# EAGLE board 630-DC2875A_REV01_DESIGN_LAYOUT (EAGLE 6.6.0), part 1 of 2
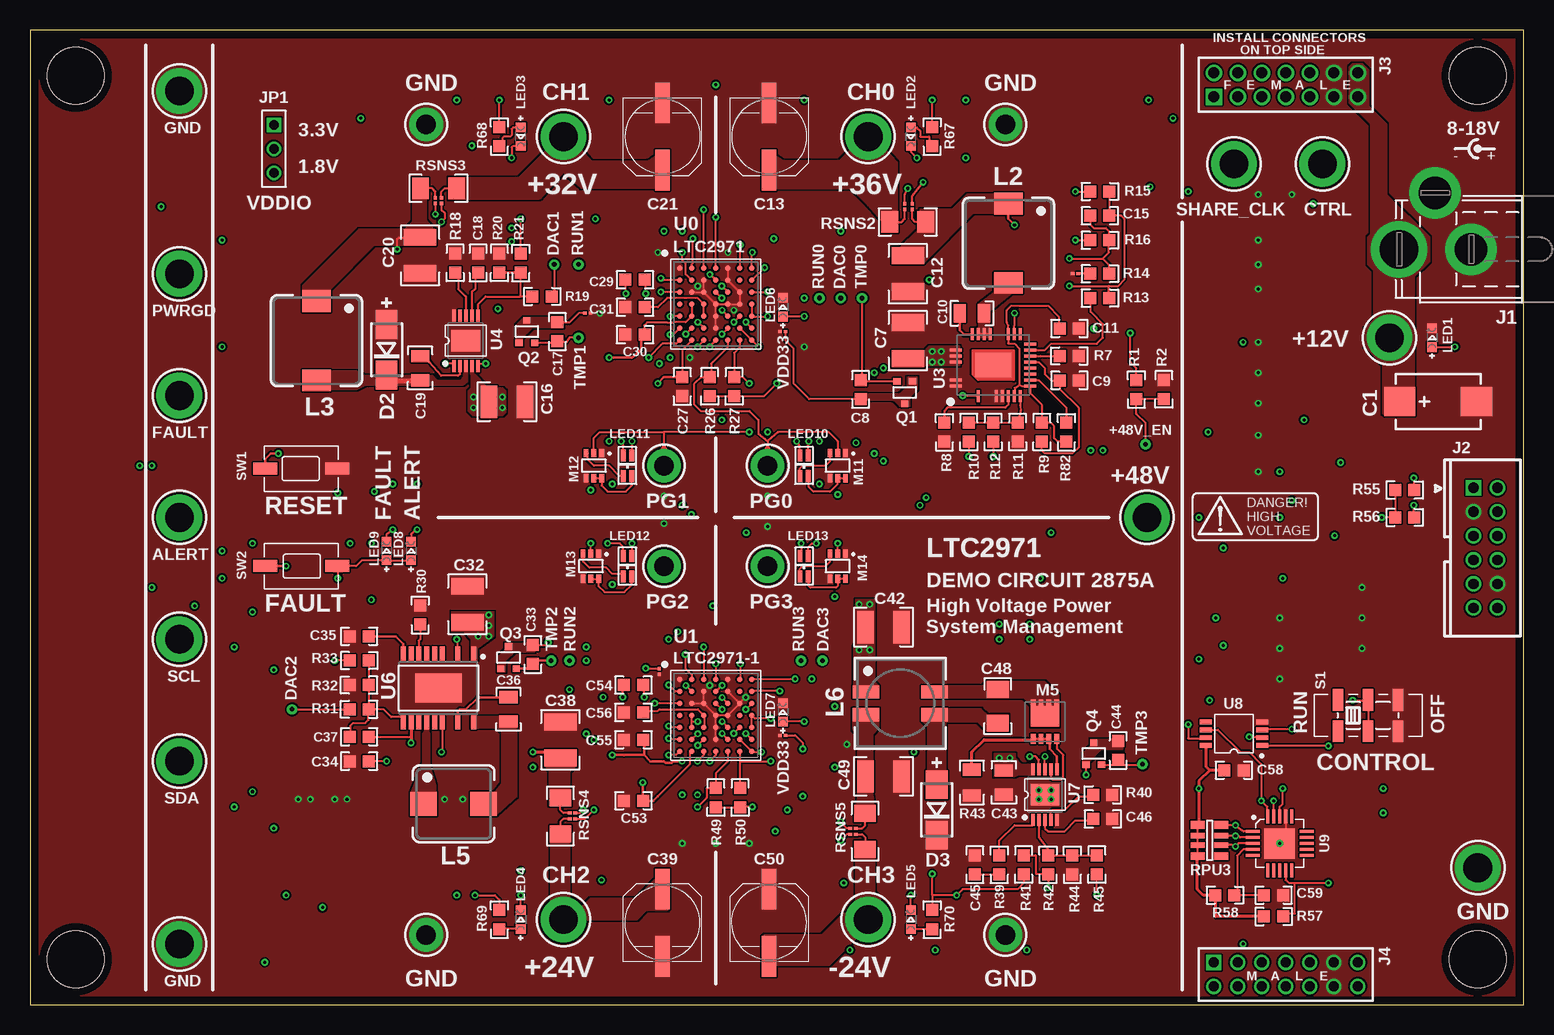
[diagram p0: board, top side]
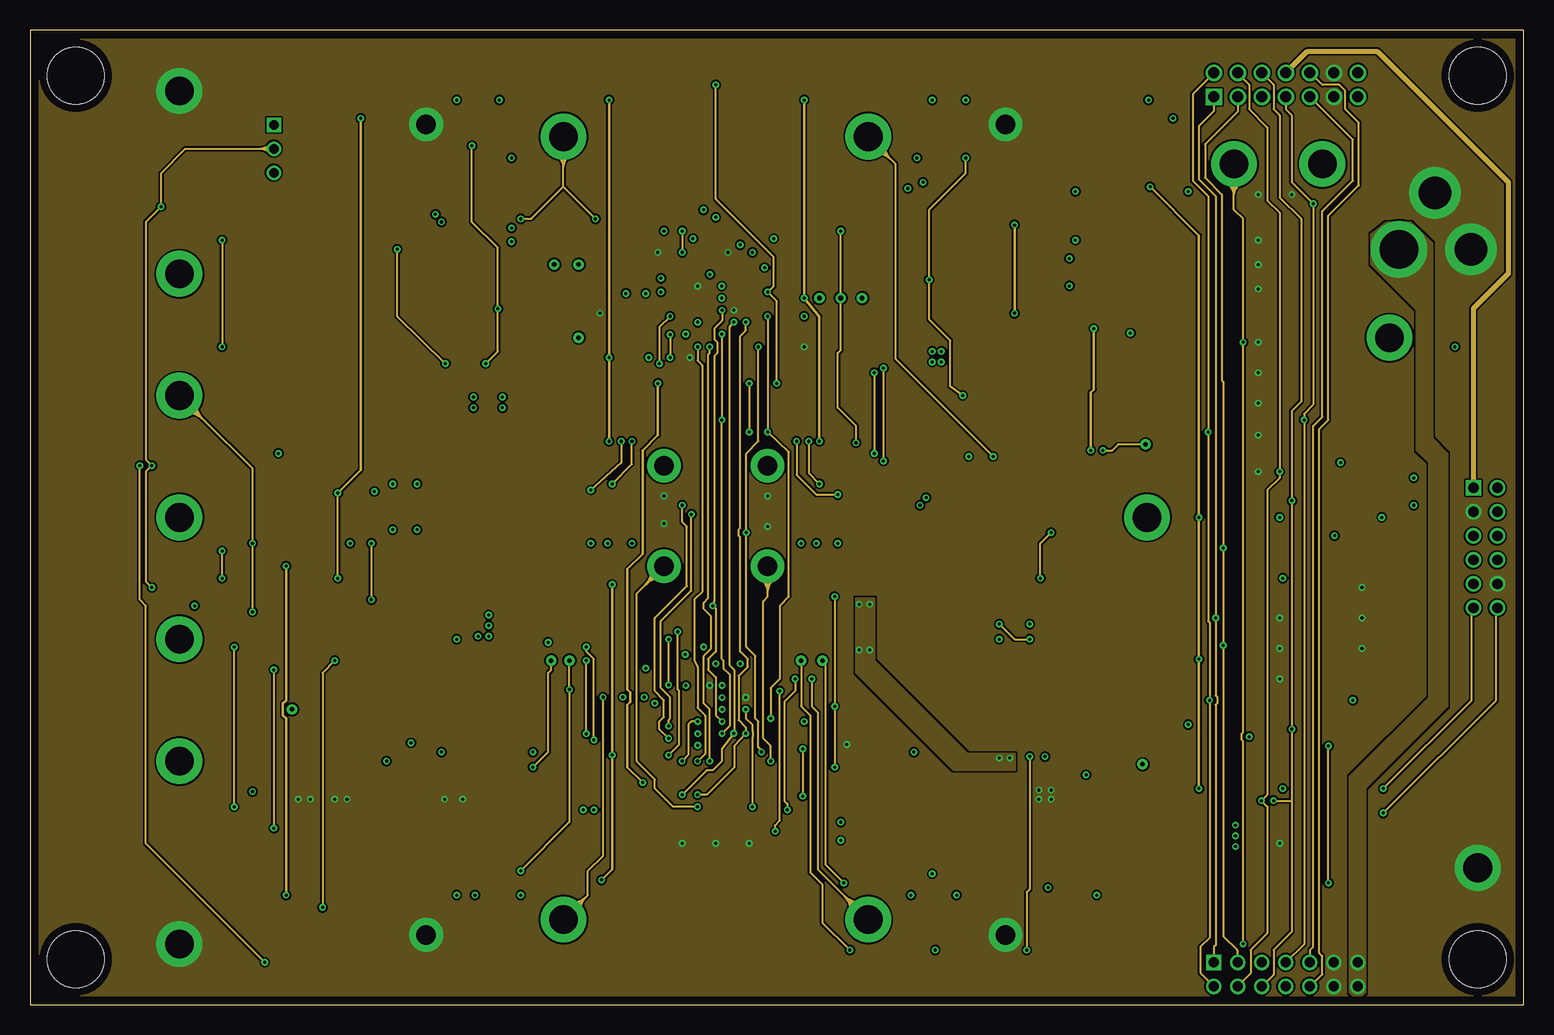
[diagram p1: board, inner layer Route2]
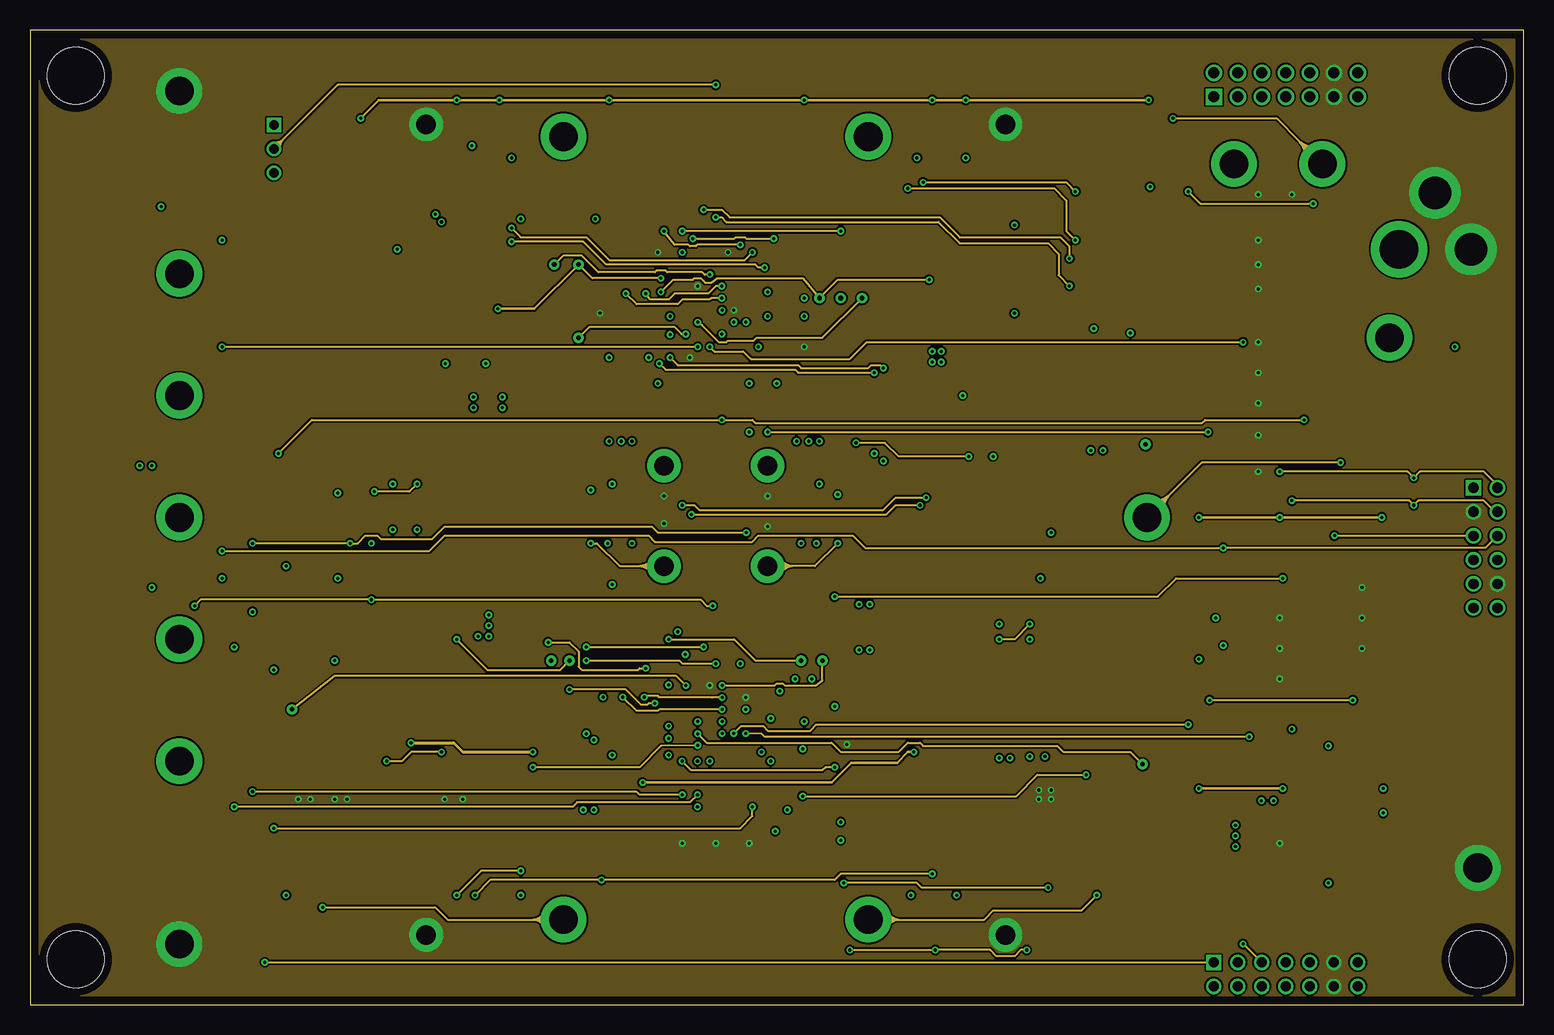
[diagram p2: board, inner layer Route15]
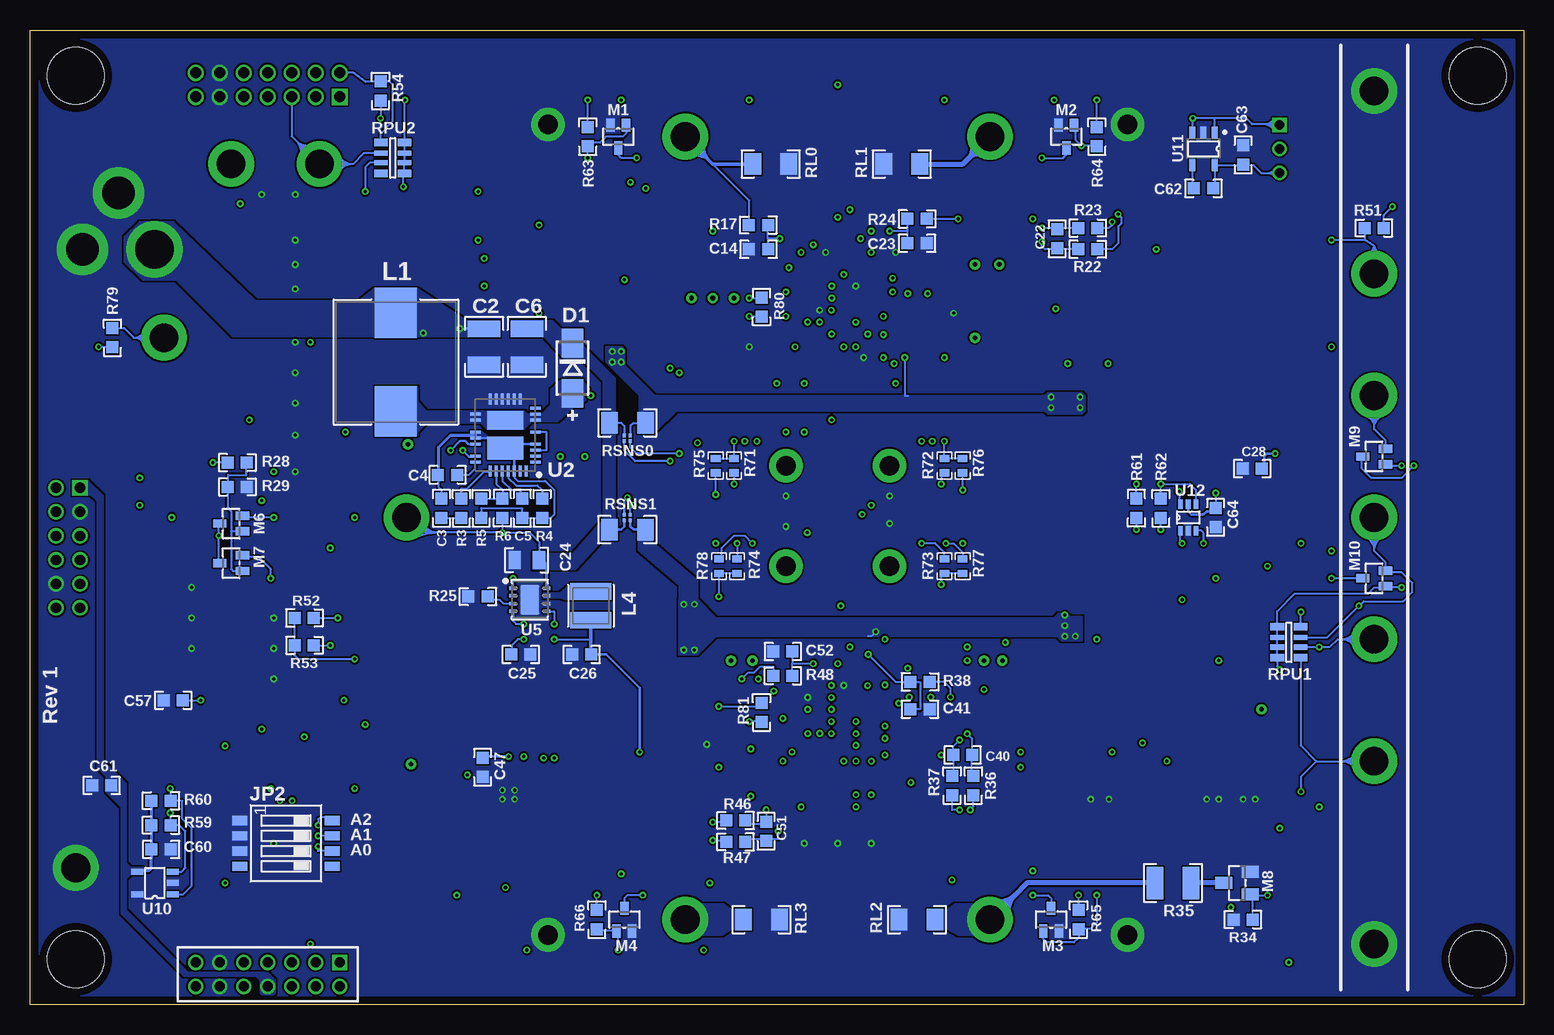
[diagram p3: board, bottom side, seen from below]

Size 124.46 x 81.28 mm. Coordinates in mm from the lower left corner, seen from the top.
Outline: 0,0 124.46,0 124.46,81.28 0,81.28 0,0
Copper layers (1*2+15*16): Top 0.035mm / dielectric 0.11mm / Route2 0.035mm / dielectric 1.13mm / Route15 0.035mm / dielectric 0.11mm / Bottom 0.035mm
Design rules "default *": minimum track width 6mil, minimum drill 10mil, track to track 6mil, track to pad 6mil, pad to pad 6mil, via to via 6mil, smd to smd 4mil, copper to edge 25mil, drill to drill 20mil, minimum pad ring 6mil, minimum via ring 6mil, stop-mask expansion 4mil, vias tented up to drill 15mil, thermal gap 10mil
Net classes: 1 HV: clearance 0.178 mm
Holes 4.75 mm at 3.81,3.81 3.81,77.47 120.65,77.47 120.65,3.81

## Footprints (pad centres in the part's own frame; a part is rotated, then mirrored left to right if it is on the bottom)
C7343 = smd 2.6 x 2.4: + -3.2,0; - 3.2,0
C1210_BOX = smd 1.4 x 2.7: 1 -1.5,0; 2 1.5,0
C0603_BOX = smd 1 x 1: 1 -0.8,0; 2 0.8,0
C0805_BOX = smd 1.016 x 1.524: 1 -1.016,0; 2 1.016,0
UD-6,3X5,8_NICHICON = smd 3.4 x 1.2: + 2.8,0; - -2.8,0
C1206_BOX = smd 1.4 x 1.8: 1 -1.4,0; 2 1.4,0
SMA = smd 2.4 x 1.8: A 2.1,0; C -2.1,0
PJ-002A/B = drill 3.2 pad 4.7: 1 3,0 | drill 2.7 pad 4.3: 2 -3,0; 3 0,-4.7
CONN_DC1613 = drill 0.86 square: 1 -5,-1 | drill 0.86: 2 -5,1; 3 -3,-1; 4 -3,1; 5 -1,-1; 6 -1,1; 7 1,-1; 8 1,1; 9 3,-1; 10 3,1; 11 5,-1; 12 5,1
2X07M = drill 0.914 square: 1 -6,-1 | drill 0.914: 2 -6,1; 3 -4,-1; 4 -4,1; 5 -2,-1; 6 -2,1; 7 0,-1; 8 0,1; 9 2,-1; 10 2,1; 11 4,-1; 12 4,1; 13 6,-1; 14 6,1
2X07M' = drill 0.85 square: 1 -6,-1 | drill 0.85: 2 -6,1; 3 -4,-1; 4 -4,1; 5 -2,-1; 6 -2,1; 7 0,-1; 8 0,1; 9 2,-1; 10 2,1; 11 4,-1; 12 4,1; 13 6,-1; 14 6,1
1X03-2MM = drill 0.8 square: 1 -2,0 | drill 0.8: 2 0,0; 3 2,0
SMT_DIP_4 = smd 1.27 x 0.762: 1 -3.861,1.905; 2 -3.861,0.635; 3 -3.861,-0.635; 4 -3.861,-1.905; 5 3.861,-1.905; 6 3.861,-0.635; 7 3.861,0.635; 8 3.861,1.905
WE-LHMI-10 = smd 4.2 x 3.5: 1 -4.1,0; 2 4.1,0
WE-PD-7.3 = smd 1.8 x 2.4: 1 3.3,0; 2 -3.3,0
WE-MAPI-3015 = smd 1.4 x 3.4: 1 -1.2,0; 2 1.2,0
WE-PD-6.0 = smd 2.2 x 2: 1 2.5,0; 2 -2.5,0
WE-DD-7.3 = smd 2.2 x 1.1: 1 -2.85,0.95; 2 -2.85,-0.95; 3 2.85,-0.95; 4 2.85,0.95
CHIPLED_0603 = smd 0.8 x 0.8: A -0.78,0; C 0.78,0
LED-DUAL_1.6X0.8MM = smd 1 x 0.4: 1 0.85,-0.35; 2 -0.85,-0.35; 3 0.85,0.35; 4 -0.85,0.35
SOT323 = smd 0.7 x 1.1: 1 -0.65,-0.95; 2 0.65,-0.95; 3 0,0.95
MLP-8 = smd 0.8 x 0.4: 1 -1.45,0.975; 2 -1.45,0.325; 3 -1.45,-0.325; 4 -1.45,-0.975 | smd 0.9 x 0.4: 5 1.4,-0.975; 6 1.4,-0.325; 7 1.4,0.325; 8 1.4,0.975 | smd 1.7 x 2.35: PAD 0.45,0
SOT23 = smd 1 x 1.4: 1 -0.95,-1.1; 2 0.95,-1.1; 3 0,1.1
SOT-363 = smd 0.7 x 0.4: 1 -1.05,0.65; 2 -1.05,0; 3 -1.05,-0.65; 4 1.05,-0.65; 5 1.05,0; 6 1.05,0.65
NODE_BREAKER = smd 0.305 x 0.254: 1 -0.229,0; 2 0.229,0
NODE_BREAKER_BOT = smd 0.305 x 0.254: 1 -0.229,0; 2 0.229,0
SC70 = smd 0.6 x 0.55: 1 -0.65,-0.925; 2 0.65,-0.925; 3 0,0.925
R0603_BOX = smd 1 x 1: 1 -0.8,0; 2 0.8,0
R1210_BOX = smd 1.4 x 2.7: 1 -1.5,0; 2 1.5,0
R0805_BOX = smd 1.016 x 1.524: 1 -1.077,0; 2 1.077,0
R0402_BOX = smd 0.6 x 0.8: 1 -0.6,0; 2 0.6,0
R1206_BOX = smd 1.4 x 1.8: 1 -1.5,0; 2 1.5,0
R_VISHAY_CRA06S = smd 1.15 x 0.63: R1_1 -0.975,1.295; R1_2 0.975,1.295; R4_1 -0.975,-1.295; R4_2 0.975,-1.295 | smd 1.15 x 0.44: R2_1 -0.975,0.4; R2_2 0.975,0.4; R3_1 -0.975,-0.4; R3_2 0.975,-0.4
JCQN = smd 0.9 x 1.8: 1 -2.5,1.3; 2 0,1.3; 3 2.5,1.3; 4 -2.5,-1.3; 5 0,-1.3; 6 2.5,-1.3
SWITCH_PTS635 = smd 2 x 1: SW1 -3,0; SW2 3,0
TURRET_LARGE_2501 = drill 2.388 pad 3.81: TP 0,0
TURRET_SMALL_2308 = drill 1.626 pad 2.794: TP1 0,0
VIA = drill 0.381 pad 0.864: 1 0,0
BGA49 = smd 0.47 x 0.47: A1 -3,3; A2 -2,3; A3 -1,3; A4 0,3; A5 1,3; A6 2,3; A7 3,3; B1 -3,2; B2 -2,2; B3 -1,2; B4 0,2; B5 1,2; B6 2,2; B7 3,2; C1 -3,1; C2 -2,1; C3 -1,1; C4 0,1; C5 1,1; C6 2,1; C7 3,1; D1 -3,0; D2 -2,0; D3 -1,0; D4 0,0; D5 1,0; D6 2,0; D7 3,0; E1 -3,-1; E2 -2,-1; E3 -1,-1; E4 0,-1; E5 1,-1; E6 2,-1; E7 3,-1; F1 -3,-2; F2 -2,-2; F3 -1,-2; F4 0,-2; F5 1,-2; F6 2,-2; F7 3,-2; G1 -3,-3; G2 -2,-3; G3 -1,-3; G4 0,-3; G5 1,-3; G6 2,-3; G7 3,-3
QFN36-5X6 = smd 0.25 x 0.9: 1 -2.25,-2.5; 2 -1.75,-2.5; 3 -1.25,-2.5; 4 -0.75,-2.5; 6 0.25,-2.5; 8 1.25,-2.5; 9 1.75,-2.5; 10 2.25,-2.5; 20 1.75,2.5; 21 1.25,2.5; 23 0.25,2.5; 24 -0.25,2.5; 25 -0.75,2.5; 27 -1.75,2.5; 28 -2.25,2.5 | smd 0.9 x 0.25: 12 3,-1.25; 13 3,-0.75; 14 3,-0.25; 15 3,0.25; 16 3,0.75; 17 3,1.25; 30 -3,1.25; 31 -3,0.75; 32 -3,0.25; 33 -3,-0.25; 34 -3,-0.75; 35 -3,-1.25; 36 -3,-1.75 | smd 1.88 x 3: 37 -1.07,0 | smd 1.53 x 3: 38 1.24,0
QFN36-5X6-UHE = smd 0.25 x 1: 3 -1.25,-2.6; 6 0.25,-2.6; 7 0.75,-2.6; 8 1.25,-2.6; 9 1.75,-2.6; 10 2.25,-2.6; 19 2.25,2.6; 20 1.75,2.6; 21 1.25,2.6; 24 -0.25,2.6; 25 -0.75,2.6; 26 -1.25,2.6; 27 -1.75,2.6 | smd 1 x 0.25: 11 3.1,-1.75; 12 3.1,-1.25; 13 3.1,-0.75; 14 3.1,-0.25; 15 3.1,0.25; 16 3.1,0.75; 17 3.1,1.25; 18 3.1,1.75; 30 -3.1,1.25; 31 -3.1,0.75; 32 -3.1,0.25; 35 -3.1,-1.25; 36 -3.1,-1.75 | smd 3 x 2: 37 0,0
MSOP10_EXP = smd 0.3 x 1: 1 -1,-2.1; 2 -0.5,-2.1; 3 0,-2.1; 4 0.5,-2.1; 5 1,-2.1; 6 1,2.1; 7 0.5,2.1; 8 0,2.1; 9 -0.5,2.1; 10 -1,2.1 | smd 2.4 x 1.8: PAD 0,0
LFCSP8 = smd 0.3 x 0.7: 1 -0.975,-1.4; 2 -0.325,-1.4; 3 0.325,-1.4; 4 0.975,-1.4; 5 0.975,1.4; 6 0.325,1.4; 7 -0.325,1.4; 8 -0.975,1.4 | smd 2.42 x 1.56: EXP 0,0
TSSOP20EXP_HV = smd 1.2 x 0.42: 1 -2.85,2.925; 3 -2.85,1.625; 5 -2.85,0.325; 6 -2.85,-0.325; 7 -2.85,-0.975; 8 -2.85,-1.625; 9 -2.85,-2.275; 10 -2.85,-2.925; 11 2.85,-2.925; 12 2.85,-2.275; 13 2.85,-1.625; 14 2.85,-0.975; 15 2.85,-0.325; 16 2.85,0.325; 18 2.85,1.625; 20 2.85,2.925 | smd 2.4 x 3.86: EXP 0,0
MSOP-8 = smd 0.406 x 1.016: 1 -0.975,-2.35; 2 -0.325,-2.35; 3 0.325,-2.35; 4 0.975,-2.35; 5 0.975,2.35; 6 0.325,2.35; 7 -0.325,2.35; 8 -0.975,2.35
QFN20 = smd 1.143 x 0.254: 1 -2.25,1; 2 -2.25,0.5; 3 -2.25,0; 4 -2.25,-0.5; 5 -2.25,-1; 11 2.25,-1; 12 2.25,-0.5; 13 2.25,0; 14 2.25,0.5; 15 2.25,1 | smd 0.254 x 1.143: 6 -1,-2.25; 7 -0.5,-2.25; 8 0,-2.25; 9 0.5,-2.25; 10 1,-2.25; 16 1,2.25; 17 0.5,2.25; 18 0,2.25; 19 -0.5,2.25; 20 -1,2.25 | smd 2.54 x 2.54: PAD 0,0
SOT-23-5 = smd 1 x 0.5: 1 -1.491,0.95; 2 -1.491,0; 3 -1.491,-0.95; 4 1.491,-0.95; 5 1.491,0.95
SOT-23-5' = smd 1 x 0.5: 1 -1.35,0.95; 2 -1.35,0; 3 -1.35,-0.95; 4 1.35,-0.95; 5 1.35,0.95
SC70-6 = smd 0.4 x 0.8: 1 -0.65,-1.102; 2 0,-1.102; 3 0.65,-1.102; 4 0.65,1.102; 5 0,1.098; 6 -0.65,1.102

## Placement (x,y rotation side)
C1  22uF/25V  [C7343]  117.35,50.29 0 top
C2  10uF/25V  [C1210_BOX]  86.61,54.86 270 bottom
C3  4.7nF  [C0603_BOX]  90.17,41.4 90 bottom
C4  4.7uF  [C0603_BOX]  89.66,44.2 180 bottom
C5  47nF  [C0603_BOX]  83.44,41.4 270 bottom
C6  4.7uF/63V  [C1210_BOX]  83.06,54.86 270 bottom
C7  4.7uF/63V  [C1210_BOX]  73.15,55.37 90 top
C8  0.1uF  [C0603_BOX]  69.22,51.31 270 top
C9  47nF  [C0603_BOX]  86.61,52.07 0 top
C10  0.1uF/63V  [C0805_BOX]  78.49,57.66 0 top
C11  1uF  [C0603_BOX]  86.61,56.39 0 top
C12  10uF/50V  [C1210_BOX]  73.15,60.96 270 top
C13  10uF/50V  [UD-6,3X5,8_NICHICON]  61.59,72.39 270 top
C14  47nF/50V  [C0603_BOX]  63.75,62.99 180 bottom
C15  0.1uF  [C0603_BOX]  89.15,65.79 180 top
C16  4.7uF/63V  [C1210_BOX]  39.75,50.29 0 top
C17  0.1uF  [C0603_BOX]  43.94,56.13 90 top
C18  47nF  [C0603_BOX]  37.34,61.85 90 top
C19  0.22uF/63V  [C0805_BOX]  32.51,53.09 270 top
C20  10uF/50V  [C1210_BOX]  32.51,62.48 270 top
C21  10uF/50V  [UD-6,3X5,8_NICHICON]  52.7,72.39 270 top
C22  0.1uF  [C0603_BOX]  38.86,63.88 90 bottom
C23  47nF/50V  [C0603_BOX]  50.55,63.5 0 bottom
C24  1uF/63V  [C0805_BOX]  83.06,37.08 180 bottom
C25  2.2nF  [C0603_BOX]  83.57,29.21 0 bottom
C26  4.7uF/10V  [C0603_BOX]  78.49,29.21 180 bottom
C27  0.1uF  [C0603_BOX]  54.36,51.56 90 top
C28  10nF  [C0603_BOX]  22.61,44.7 0 bottom
C29  0.1uF  [C0603_BOX]  50.42,60.45 180 top
C30  0.1uF  [C0603_BOX]  50.42,55.88 180 top
C31  0.1uF  [C0603_BOX]  50.42,58.17 0 top
C32  4.7uF/63V  [C1210_BOX]  36.45,33.4 90 top
C33  0.1uF  [C0603_BOX]  41.91,29.21 90 top
C34  4.7uF/10V  [C0603_BOX]  27.43,20.32 180 top
C35  47nF  [C0603_BOX]  27.43,30.73 180 top
C36  0.1uF/63V  [C0805_BOX]  39.88,24.64 270 top
C37  22pF  [C0603_BOX]  27.43,22.35 180 top
C38  10uF/35V  [C1210_BOX]  44.2,22.1 90 top
C39  10uF/35V  [UD-6,3X5,8_NICHICON]  52.7,6.86 90 top
C40  0.1uF  [C0603_BOX]  46.74,20.83 180 bottom
C41  47nF/50V  [C0603_BOX]  50.29,24.64 0 bottom
C42  4.7uF/63V  [C1210_BOX]  71.12,31.5 0 top
C43  0.1uF/63V  [C0805_BOX]  81.15,18.54 270 top
C44  0.1uF  [C0603_BOX]  90.68,21.21 90 top
C45  4.7nF  [C0603_BOX]  78.74,11.68 90 top
C46  220nF  [C0603_BOX]  89.41,15.49 0 top
C47  4.7uF/10V  [C0603_BOX]  86.74,19.81 270 bottom
C48  2.2uF/100V  [C1206_BOX]  80.64,24.89 270 top
C49  10uF/35V  [C1210_BOX]  71.12,19.05 0 top
C50  10uF/35V  [UD-6,3X5,8_NICHICON]  61.59,6.86 90 top
C51  0.1uF  [C0603_BOX]  63.12,14.48 270 bottom
C52  47nF/50V  [C0603_BOX]  61.72,29.46 180 bottom
C53  0.1uF  [C0603_BOX]  50.29,17.02 180 top
C54  0.1uF  [C0603_BOX]  50.29,26.67 180 top
C55  0.1uF  [C0603_BOX]  50.29,22.1 180 top
C56  0.1uF  [C0603_BOX]  50.29,24.38 180 top
C57  1uF  [C0603_BOX]  112.52,25.4 180 bottom
C58  0.1uF  [C0603_BOX]  100.33,19.56 0 top
C59  1uF  [C0603_BOX]  103.63,9.14 0 top
C60  0.1uF  [C0603_BOX]  113.54,12.95 0 bottom
C61  1uF/10V  [C0603_BOX]  118.49,18.29 180 bottom
C62  10nF  [C0603_BOX]  26.67,68.07 180 bottom
C63  4.7uF/10V  [C0603_BOX]  23.37,70.87 90 bottom
C64  0.1uF  [C0603_BOX]  25.65,40.64 270 bottom
D1  B160-13-F  [SMA]  79.25,53.09 270 bottom
D2  B160-13-F  [SMA]  29.72,54.61 90 top
D3  B160-13-F  [SMA]  75.56,16.26 90 top
DRILEGEND  [DRILEGEND]  not placed on the board
J1  PJ-002A  [PJ-002A/B]  117.09,62.99 180 top
J2  [CONN_DC1613]  121.28,38.1 270 top
J3  FEMALE  [2X07M]  104.65,76.71 0 top
J4  MALE  [2X07M']  104.65,2.54 180 bottom
JP1  [1X03-2MM]  20.32,71.37 270 top
JP2  TDA04H0SK1  [SMT_DIP_4]  103.12,13.46 0 bottom
L1  33uH  [WE-LHMI-10]  93.98,53.59 270 bottom
L2  47uH  [WE-PD-7.3]  81.53,63.5 270 top
L3  47uH  [WE-PD-7.3]  23.88,55.37 270 top
L4  33uH  [WE-MAPI-3015]  77.72,33.27 270 bottom
L5  33uH  [WE-PD-6.0]  35.31,16.76 0 top
L6  100uH  [WE-DD-7.3]  72.52,25.15 0 top
LED1  BLUE  [CHIPLED_0603]  116.84,55.63 90 top
LED2  GREEN  [CHIPLED_0603]  73.41,72.39 270 top
LED3  GREEN  [CHIPLED_0603]  40.89,72.39 270 top
LED4  GREEN  [CHIPLED_0603]  40.89,7.11 90 top
LED5  GREEN  [CHIPLED_0603]  73.41,7.11 90 top
LED6  GREEN  [CHIPLED_0603]  62.74,58.17 90 top
LED7  GREEN  [CHIPLED_0603]  62.74,24.38 90 top
LED8  RED  [CHIPLED_0603]  31.75,37.85 90 top
LED9  RED  [CHIPLED_0603]  29.72,37.85 90 top
LED10  LED-DUAL-COLOR-BL-RD  [LED-DUAL_1.6X0.8MM]  64.52,44.96 90 top
LED11  LED-DUAL-COLOR-BL-RD  [LED-DUAL_1.6X0.8MM]  49.78,44.96 90 top
LED12  LED-DUAL-COLOR-BL-RD  [LED-DUAL_1.6X0.8MM]  49.78,36.58 90 top
LED13  LED-DUAL-COLOR-BL-RD  [LED-DUAL_1.6X0.8MM]  64.52,36.58 90 top
M1  DMG1012UW-7  [SOT323]  75.44,72.39 180 bottom
M2  DMG1012UW-7  [SOT323]  38.1,72.39 180 bottom
M3  DMG1012UW-7  [SOT323]  39.37,7.11 0 bottom
M4  DMG1012UW-7  [SOT323]  74.93,7.11 0 bottom
M5  FDMC86102L  [MLP-8]  84.58,23.62 90 top
M6  NTS4173P  [SOT323]  107.7,40.13 90 bottom
M7  NTS4173P  [SOT323]  107.7,36.83 90 bottom
M8  DMN6140L  [SOT23]  23.88,10.16 90 bottom
M9  BSS138  [SOT323]  12.45,45.72 90 bottom
M10  BSS138  [SOT323]  12.45,35.56 90 bottom
M11  DMN63D8LDW  [SOT-363]  67.31,44.96 270 top
M12  DMN63D8LDW  [SOT-363]  46.99,44.96 270 top
M13  DMN63D8LDW  [SOT-363]  46.74,36.58 270 top
M14  DMN63D8LDW  [SOT-363]  67.31,36.58 270 top
NB1  NODE_BREAKER  [NODE_BREAKER]  45.21,16 0 top
NB2  NODE_BREAKER  [NODE_BREAKER]  45.21,15.49 0 top
NB3  NODE_BREAKER  [NODE_BREAKER]  33.78,67.06 270 top
NB4  NODE_BREAKER  [NODE_BREAKER]  34.29,67.06 270 top
NB5  NODE_BREAKER  [NODE_BREAKER]  62.74,56.13 0 top
NB6  NODE_BREAKER  [NODE_BREAKER]  68.58,14.73 180 top
NB7  NODE_BREAKER  [NODE_BREAKER]  68.58,14.22 180 top
NB12  NODE_BREAKER_BOT  [NODE_BREAKER_BOT]  74.93,47.24 270 bottom
NB13  NODE_BREAKER_BOT  [NODE_BREAKER_BOT]  74.42,47.24 270 bottom
NB14  NODE_BREAKER  [NODE_BREAKER]  46.48,57.66 180 top
NB15  NODE_BREAKER  [NODE_BREAKER]  52.45,27.81 90 top
NB16  NODE_BREAKER  [NODE_BREAKER]  62.74,22.48 0 top
NB17  NODE_BREAKER_BOT  [NODE_BREAKER_BOT]  74.93,40.64 90 bottom
NB18  NODE_BREAKER_BOT  [NODE_BREAKER_BOT]  74.42,40.64 90 bottom
NB19  NODE_BREAKER  [NODE_BREAKER]  87.12,60.96 180 top
NB20  NODE_BREAKER  [NODE_BREAKER]  73.53,66.55 270 top
NB21  NODE_BREAKER  [NODE_BREAKER]  72.9,66.55 270 top
Q1  MMBT3906  [SC70]  72.9,51.05 180 top
Q2  MMBT3906  [SC70]  41.4,56.13 0 top
Q3  MMBT3906  [SC70]  39.88,28.96 0 top
Q4  MMBT3906  [SC70]  88.65,20.95 0 top
R1  49.9k  [R0603_BOX]  92.2,51.31 90 top
R2  10k  [R0603_BOX]  94.49,51.31 270 top
R3  15k  [R0603_BOX]  88.52,41.4 90 bottom
R4  41.2k  [R0603_BOX]  81.79,41.4 90 bottom
R5  10k  [R0603_BOX]  86.87,41.4 90 bottom
R6  294k  [R0603_BOX]  85.09,41.4 270 bottom
R7  41.2k  [R0603_BOX]  86.61,54.1 180 top
R8  6.49k  [R0603_BOX]  76.2,47.75 90 top
R9  75k  [R0603_BOX]  84.33,47.75 270 top
R10  200k  [R0603_BOX]  78.23,47.75 270 top
R11  10k  [R0603_BOX]  82.3,47.75 270 top
R12  348k  [R0603_BOX]  80.26,47.75 270 top
R13  0R  [R0603_BOX]  89.15,58.93 0 top
R14  0R  [R0603_BOX]  89.15,60.96 0 top
R15  200  [R0603_BOX]  89.15,67.82 0 top
R16  200  [R0603_BOX]  89.15,63.75 0 top
R17  200  [R0603_BOX]  63.75,65.02 180 bottom
R18  60.4k  [R0603_BOX]  35.43,61.85 270 top
R19  200k  [R0603_BOX]  42.67,59.05 0 top
R20  10k  [R0603_BOX]  39.12,61.85 270 top
R21  261k  [R0603_BOX]  40.89,61.85 90 top
R22  200  [R0603_BOX]  36.32,62.99 0 bottom
R23  200  [R0603_BOX]  36.32,64.77 0 bottom
R24  200  [R0603_BOX]  50.55,65.53 0 bottom
R25  1k  [R0603_BOX]  87.12,34.04 180 bottom
R26  10k  [R0603_BOX]  56.64,51.56 270 top
R27  10k  [R0603_BOX]  58.67,51.56 270 top
R28  499k  [R0603_BOX]  107.19,45.21 0 bottom
R29  100k  [R0603_BOX]  107.19,43.18 0 bottom
R30  8.66k  [R0603_BOX]  32.51,32.51 90 top
R31  124k  [R0603_BOX]  27.43,24.64 180 top
R32  10k  [R0603_BOX]  27.43,26.67 180 top
R33  287k  [R0603_BOX]  27.43,28.7 0 top
R34  100k  [R0603_BOX]  23.37,7.11 180 bottom
R35  20  [R1210_BOX]  29.21,10.16 180 bottom
R36  200  [R0603_BOX]  45.85,18.29 90 bottom
R37  200  [R0603_BOX]  47.62,18.29 90 bottom
R38  200  [R0603_BOX]  50.29,26.92 0 bottom
R39  15k  [R0603_BOX]  80.77,11.68 90 top
R40  41.2k  [R0603_BOX]  89.41,17.53 180 top
R41  210k  [R0603_BOX]  82.8,11.68 270 top
R42  200k  [R0603_BOX]  84.84,11.68 90 top
R43  0.015  [R0805_BOX]  78.49,18.54 90 top
R44  10k  [R0603_BOX]  86.87,11.68 90 top
R45  261k  [R0603_BOX]  88.9,11.68 270 top
R46  200  [R0603_BOX]  65.66,15.37 180 bottom
R47  200  [R0603_BOX]  65.66,13.59 180 bottom
R48  200  [R0603_BOX]  61.72,27.43 180 bottom
R49  10k  [R0603_BOX]  57.15,17.27 270 top
R50  10k  [R0603_BOX]  59.18,17.27 270 top
R51  10k  [R0603_BOX]  12.45,64.77 180 bottom
R52  10k  [R0603_BOX]  101.6,32.26 0 bottom
R53  10k  [R0603_BOX]  101.6,29.97 0 bottom
R54  1k  [R0603_BOX]  95.25,76.2 90 bottom
R55  10k  [R0603_BOX]  114.55,42.93 0 top
R56  10k  [R0603_BOX]  114.55,40.64 0 top
R57  10k  [R0603_BOX]  103.63,7.37 0 top
R58  249  [R0603_BOX]  99.57,9.14 0 top
R59  10k  [R0603_BOX]  113.54,14.99 180 bottom
R60  10k  [R0603_BOX]  113.54,17.02 180 bottom
R61  698  [R0603_BOX]  32.26,41.4 270 bottom
R62  698  [R0603_BOX]  30.23,41.4 90 bottom
R63  10k  [R0603_BOX]  77.98,72.39 90 bottom
R64  10k  [R0603_BOX]  35.56,72.39 90 bottom
R65  10k  [R0603_BOX]  37.08,7.11 90 bottom
R66  10k  [R0603_BOX]  77.22,7.11 90 bottom
R67  15k  [R0603_BOX]  75.18,72.39 90 top
R68  15k  [R0603_BOX]  39.12,72.39 90 top
R69  15k  [R0603_BOX]  39.12,7.11 90 top
R70  15k  [R0603_BOX]  75.18,7.11 90 top
R71  3k  [R0402_BOX]  65.79,44.96 90 bottom
R72  3k  [R0402_BOX]  48.26,44.96 90 bottom
R73  3k  [R0402_BOX]  48.26,36.58 270 bottom
R74  3k  [R0402_BOX]  65.53,36.58 270 bottom
R75  1k  [R0402_BOX]  67.31,44.96 90 bottom
R76  1k  [R0402_BOX]  46.74,44.96 90 bottom
R77  1k  [R0402_BOX]  46.74,36.58 270 bottom
R78  1k  [R0402_BOX]  67.06,36.58 270 bottom
R79  40.2k  [R0603_BOX]  117.6,55.63 90 bottom
R80  15k  [R0603_BOX]  63.5,58.17 270 bottom
R81  15k  [R0603_BOX]  63.5,24.38 90 bottom
R82  0R  [R0603_BOX]  86.36,47.75 90 top
RL0  7.15k  [R1206_BOX]  62.74,70.1 180 bottom
RL1  6.34k  [R1206_BOX]  51.82,70.1 0 bottom
RL2  4.75k  [R1206_BOX]  50.55,7.11 0 bottom
RL3  4.75k  [R1206_BOX]  63.5,7.11 180 bottom
RPU1  10k, 4X  [R_VISHAY_CRA06S]  19.56,30.23 180 bottom
RPU2  10k, 4X  [R_VISHAY_CRA06S]  94.23,70.61 0 bottom
RPU3  10k, 4X  [R_VISHAY_CRA06S]  98.3,13.72 180 top
RSNS0  0.05  [R1206_BOX]  74.68,48.51 0 bottom
RSNS1  0.05  [R1206_BOX]  74.68,39.62 0 bottom
RSNS2  0.05  [R1206_BOX]  73.15,65.28 180 top
RSNS3  0.05  [R1206_BOX]  34.04,68.07 0 top
RSNS4  0.05  [R1206_BOX]  44.2,15.75 270 top
RSNS5  0.05  [R1206_BOX]  69.6,14.48 270 top
S1  JS202011JCQN  [JCQN]  111.51,24.13 0 top
SW1  RS-282G05A3-SM RT  [SWITCH_PTS635]  22.61,44.7 0 top
SW2  RS-282G05A3-SM RT  [SWITCH_PTS635]  22.61,36.58 180 top
TP0  CH0  [TURRET_LARGE_2501]  69.85,72.39 0 top
TP1  CH1  [TURRET_LARGE_2501]  44.45,72.39 0 top
TP2  CH2  [TURRET_LARGE_2501]  44.45,7.11 0 top
TP3  CH3  [TURRET_LARGE_2501]  69.85,7.11 0 top
TP4  PWRGD  [TURRET_LARGE_2501]  12.45,60.96 0 top
TP5  FAULT  [TURRET_LARGE_2501]  12.45,50.8 0 top
TP6  ALERT  [TURRET_LARGE_2501]  12.45,40.64 0 top
TP7  SCL  [TURRET_LARGE_2501]  12.45,30.48 0 top
TP8  SDA  [TURRET_LARGE_2501]  12.45,20.32 0 top
TP9  GND  [TURRET_LARGE_2501]  12.45,76.2 0 top
TP10  GND  [TURRET_LARGE_2501]  120.65,11.43 0 top
TP11  GND  [TURRET_LARGE_2501]  12.45,5.08 0 top
TP12  SHARE_CLK  [TURRET_LARGE_2501]  100.33,70.1 0 top
TP13  CTRL  [TURRET_LARGE_2501]  107.7,70.1 0 top
TP14  +12V  [TURRET_LARGE_2501]  113.28,55.63 0 top
TP15  +48V  [TURRET_LARGE_2501]  93.09,40.64 0 top
TP16  PG1  [TURRET_SMALL_2308]  61.47,44.96 0 top
TP17  PG0  [TURRET_SMALL_2308]  52.83,44.96 0 top
TP18  PG2  [TURRET_SMALL_2308]  52.83,36.58 0 top
TP19  PG3  [TURRET_SMALL_2308]  61.47,36.58 0 top
TP20  [TURRET_SMALL_2308]  81.28,73.41 0 top
TP21  [TURRET_SMALL_2308]  33.02,73.41 0 top
TP22  [TURRET_SMALL_2308]  33.02,5.84 0 top
TP23  [TURRET_SMALL_2308]  81.28,5.84 0 top
TP24  TESPOINT_SMD  [VIA]  65.79,58.93 0 top
TP25  TESPOINT_SMD  [VIA]  69.34,58.93 0 top
TP26  TESPOINT_SMD  [VIA]  67.56,58.93 0 top
TP27  TESPOINT_SMD  [VIA]  45.72,61.72 0 top
TP28  TESPOINT_SMD  [VIA]  45.72,55.63 0 top
TP29  TESPOINT_SMD  [VIA]  43.69,61.72 0 top
TP30  TESTPOINT_SMD  [VIA]  44.96,28.7 0 top
TP31  TESPOINT_SMD  [VIA]  43.43,28.7 0 top
TP32  TESPOINT_SMD  [VIA]  21.84,24.64 0 top
TP33  TESPOINT_SMD  [VIA]  64.26,28.7 0 top
TP34  TESPOINT_SMD  [VIA]  92.71,20.07 270 top
TP35  TESPOINT_SMD  [VIA]  66.04,28.7 0 top
TP36  TESPOINT_SMD  [VIA]  92.96,46.74 0 top
U0  LTC2971  [BGA49]  57.15,58.42 0 top
U1  LTC2971-1  [BGA49]  57.15,24.13 0 top
U2  LT3958  [QFN36-5X6]  84.84,47.5 90 bottom
U3  LT7101  [QFN36-5X6-UHE]  80.26,53.34 0 top
U4  LT3991  [MSOP10_EXP]  36.32,55.37 0 top
U5  ADP2360-5.0  [LFCSP8]  82.8,33.78 270 bottom
U6  LT8630  [TSSOP20EXP_HV]  34.04,26.42 270 top
U7  LT3758  [MSOP10_EXP]  84.58,17.53 0 top
U8  LTC4313-3  [MSOP-8]  100.33,22.61 90 top
U9  MCP23008-E/ML  [QFN20]  104.14,13.46 0 top
U10  24AA02T-I/OT  [SOT-23-5]  114.05,10.16 180 bottom
U11  LT1761-1.8V  [SOT-23-5']  26.67,71.37 270 bottom
U12  SN74LVC2G34  [SC70-6]  27.94,40.64 0 bottom
U$3  [LOGO_ADI_POWER_BY_LINEAR]  6.73,9.91 90 top
U$4  [LOGO_ADI_POWER_BY_LINEAR]  2.79,9.91 90 bottom
U$59  [HV_SIGN]  102.36,40.89 0 top
U$63  [DC2875_FRAME]  not placed on the board

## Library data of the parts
C1-C64 = rcl
D1-D3 = diode
DRILEGEND = drilegend
J1 = power-jack
J2 = con-fci
J3 = pinhead_2mm
J4 = pinhead-2mm
JP1 = pinhead
JP2 SW1 SW2 U9 U10 U12 U$59 = kalin
L1-L6 = inductors
LED1-LED13 = led
M1-M14 = transistor-fet
NB1-NB7 NB12-NB21 = solderpad
Q1-Q4 = transistor-small-signal
R1-R82 RL0 RL1-RL3 RPU1-RPU3 RSNS0 RSNS1-RSNS5 = resistor
S1 = switch
TP0 TP1-TP36 = testpad
U0 U1-U4 U6-U8 U11 U$3 U$4 = linear-technology
U5 = analog-devices
U$63 = frames

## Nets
+12V: C1.+ C2.1 J1.1 J3.13 J3.14 J4.13 J4.14 L1.1 R1.2 R79.2 TP14.TP U2.27
+48V [HV]: C6.1 C24.1 D1.C NB12.1 NB17.1 R6.2 R28.1 RSNS0.1 RSNS1.1 TP15.TP U5.1 U5.8
+48V_EN: R1.1 R2.2 TP36.1 U2.25
A0_MUX: JP2.6 RPU3.R2_1 U9.3
A1_MUX: JP2.7 RPU3.R3_1 U9.2
A2_MUX: JP2.8 RPU3.R4_1 U9.1
ALERTB: M10.2 RPU1.R3_1 TP6.TP U0.E5 U1.E5 U12.1
ALERTB_3V3: J2.6 J3.3 J4.3 M10.3 R53.2
CTRL: C57.1 J3.2 J4.2 R54.2 RPU2.R1_1 S1.2 S1.5 U0.D7 U0.E7 U1.D7 U1.E7
CTRL_P: R54.1 TP13.TP
DAC_CH0: R10.2 TP26.1 U0.B2
DAC_CH1: R19.2 TP29.1 U0.B4
DAC_CH2: R31.2 TP32.1 U1.B2
DAC_CH3: R41.1 R42.1 TP35.1 U1.B4
EESCL: J2.11 R60.1 U10.1
EESDA: J2.12 R59.1 U10.3
FAULTB: M9.2 RPU1.R4_1 TP5.TP U0.F6 U0.G7 U1.F6 U1.G7 U12.3
FAULTB_3V3: J3.1 J4.1 M9.3 R52.2
GND: C1.- C2.2 C6.2 C7.2 C9.2 C11.2 C12.2 C13.- C14.2 C16.2 C18.2 C20.2 C21.- C23.2 C24.2 C25.2 C26.2 C27.1 C28.1 C30.2 C31.1 C32.2 C34.2 C35.2 C38.2 C39.- C41.2 C42.2 C43.2 C45.2 C46.2 C47.2 C49.2 C50.+ C52.2 C53.2 C55.2 C56.2 C57.2 C58.2 C59.2 C60.2 C61.2 C63.2 C64.2 D2.A D3.C J1.2 J1.3 J2.3 J2.10 J3.11 J3.12 J4.11 J4.12 JP2.1 JP2.2 JP2.3 LED1.C LED6.C LED7.C M1.2 M2.2 M3.2 M4.2 M8.2 M11.1 M11.4 M12.1 M12.4 M13.1 M13.4 M14.1 M14.4 NB5.1 NB14.1 NB15.1 NB16.1 NB19.2 R2.1 R7.1 R8.1 R11.2 R18.1 R20.1 R25.2 R29.2 R30.2 R32.2 R34.2 R40.1 R43.1 R44.1 RL0.1 RL1.1 RL2.1 RL3.1 S1.3 S1.6 SW1.SW2 TP9.TP TP10.TP TP11.TP TP20.TP1 TP21.TP1 TP22.TP1 TP23.TP1 U0.A1 U0.A5 U0.B3 U0.B5 U0.C2 U0.C3 U0.C6 U0.D4 U0.D5 U0.D6 U0.E4 U0.F4 U1.A1 U1.A5 U1.B3 U1.B5 U1.C2 U1.C3 U1.C6 U1.D4 U1.D5 U1.E4 U1.F4 U2.12 U2.13 U2.14 U2.15 U2.16 U2.17 U3.6 U3.7 U3.35 U3.36 U3.37 U4.10 U4.PAD U5.6 U5.EXP U6.EXP U7.5 U7.PAD U8.4 U9.17 U9.PAD U10.2 U10.5 U11.2 U12.2
IIN_SNSM0 [HV]: NB13.2 U0.E1
IIN_SNSM1 [HV]: NB18.2 U1.E1
IIN_SNSP0 [HV]: NB12.2 U0.F1
IIN_SNSP1 [HV]: NB17.2 U1.F1
INTVCC: C11.1 R9.1 R82.1 U3.9 U3.11 U3.21
IOUT_SNSM_CH0 [HV]: C15.2 R14.2 R16.2 U0.A3
IOUT_SNSM_CH1 [HV]: C22.2 R23.1 U0.A7
IOUT_SNSM_CH2: C40.2 R37.2 U1.A3
IOUT_SNSM_CH3: C51.1 R46.1 U1.A7
IOUT_SNSP_CH0 [HV]: C15.1 R13.2 R15.2 U0.A4
IOUT_SNSP_CH1 [HV]: C22.1 R22.1 U0.B7
IOUT_SNSP_CH2: C40.1 R36.2 U1.A4
IOUT_SNSP_CH3: C51.2 R47.1 U1.B7
N$1: R61.1 U12.6
N$2: M8.1 R34.1 SW2.SW2
N$3: LED8.C R61.2
N$4: R7.2 U3.16
N$5: LED4.C M3.3
N$6: LED2.C M1.3
N$7: LED2.A R67.1
N$8: C4.1 U2.28
N$9: LED4.A R69.1
N$10: LED3.C M2.3
N$11: LED3.A R68.1
N$12: LED1.A R79.1
N$13: U2.3 U2.6
N$14: C54.1 U1.C5
N$15: C54.2 U1.C4
N$16: LED5.A R70.1
N$17: LED5.C M4.3
N$18: R3.2 U2.30
N$19: C56.1 U1.D3 U1.E3
N$20: R8.2 U3.8
N$21: C5.1 U2.32
N$22: M5.1 M5.2 M5.3 R43.2 U7.6
N$23: C25.1 U5.5
N$24: C62.2 U11.4
N$25: R62.2 U12.4
N$26: LED9.C R62.1
N$27: C37.1 C38.1 NB1.1 RSNS4.1 U6.12
N$28: LED11.2 M12.5 M12.6
N$30 [HV]: D1.A L1.2 U2.8 U2.9 U2.20 U2.21 U2.38
N$32: R4.2 U2.33
N$33: R18.2 U4.8
N$34: M5.4 U7.7
N$35 [HV]: C36.1 U6.18
N$36 [HV]: C20.1 L3.2 NB3.1 RSNS3.1 U4.1
N$37: C34.1 U6.16
N$38: R30.1 U6.8
N$39 [HV]: C36.2 L5.1 U6.20
N$40: L5.2 U6.14
N$41: C35.1 U6.10
N$42: C46.1 U7.3
N$43 [HV]: C48.1 L6.4 M5.5 M5.6 M5.7 M5.8 M5.PAD
N$44 [HV]: C48.2 D3.A L6.3
N$45: R40.2 U7.4
N$46: L4.1 U5.7
N$47: R39.2 U7.1
N$48: R25.1 U5.3
N$49: C29.2 U0.C4
N$50: C45.1 R39.1
N$51: R5.2 R6.1 U2.31
N$52: C31.2 U0.D3 U0.E3
N$53: C29.1 U0.C5
N$54: C62.1 C63.1 JP1.3 U11.5
N$55: M8.3 R35.1
N$56: LED11.1 R72.1
N$57: LED11.4 M12.3
N$58: LED10.1 R71.1
N$59: C18.1 U4.7
N$60: LED10.3 R75.1
N$61: C3.1 R3.1
N$62: C49.1 L6.2 NB6.1 RSNS5.1
N$63: LED6.A R80.2
N$64: C8.2 NB5.2 Q1.1 Q1.3
N$65: LED7.A R81.1
N$66: C59.1 R58.2 U9.4
N$67: C17.2 NB14.2 Q2.1 Q2.3
N$68: C33.2 NB15.2 Q3.1 Q3.3
N$69: C44.2 NB16.2 Q4.1 Q4.3
N$70: C19.2 D2.C L3.1 U4.3
N$71: C19.1 U4.2
N$73: C9.1 R9.2 U3.15
N$74: R57.2 U8.1 U9.9
N$75 [HV]: R13.1 U3.17
N$77: C47.1 U7.8
N$78 [HV]: C12.1 L2.2 NB20.2 RSNS2.1 U3.20
N$82: LED10.2 M11.5 M11.6
N$83: LED11.3 R76.1
N$84: LED12.2 M13.5 M13.6
N$85: LED12.4 M13.3
N$86: LED13.2 M14.5 M14.6
N$87: LED13.4 M14.3
N$88: LED13.1 R74.1
N$89: LED13.3 R78.1
N$91: LED12.1 R73.1
N$92: LED12.3 R77.1
N$94: NB20.1 R15.1
N$96: LED10.4 M11.3
N$98 [HV]: NB19.1 R14.1
N$99: NB21.1 R16.1
N$100: C10.2 L2.1 U3.24 U3.25 U3.26
N$109: NB1.2 R36.1
N$114: C10.1 U3.27
N$116: R82.2 U3.12
N$300 [HV]: NB3.2 R22.2
N$301 [HV]: NB4.2 R23.2
N$304: NB7.2 R47.2
N$305: NB6.2 R46.2
N$500: NB2.2 R37.1
PFET_GATE: M6.1 M7.1 R28.2 R29.1
PG0: M11.2 R26.1 TP16.TP1 U0.G5
PG1: M12.2 R27.1 TP17.TP1 U0.G6
PG2: M13.2 R49.1 TP18.TP1 U1.G5
PG3: M14.2 R50.1 TP19.TP1 U1.G6
PWRGD: R51.2 TP4.TP U0.G3 U1.G3
RESETB: C28.2 J3.7 J4.7 RPU2.R3_1 SW1.SW1 U0.F5 U1.F5
RUN_CH0: M1.1 R63.1 TP24.1 U0.C1 U3.3
RUN_CH1: M2.1 R64.1 TP27.1 U0.B1 U4.5
RUN_CH2: M3.1 R65.1 TP30.1 U1.C1 U6.3
RUN_CH3: M4.1 R66.1 TP33.1 U1.B1 U7.9
SCL: RPU1.R2_1 TP7.TP U0.F7 U1.F7 U8.2
SCL_IN: J2.4 J3.6 J4.6 R56.2 U8.3 U9.19
SDA: RPU1.R1_1 TP8.TP U0.E6 U1.E6 U8.7
SDA_IN: J2.2 J3.4 J4.4 R55.2 U8.6 U9.20
SGND: C3.2 C4.2 C5.2 R4.1 R5.1 U2.4 U2.23 U2.24 U2.34 U2.37
SHARE_CLK: J3.5 J4.5 RPU2.R2_1 TP12.TP U0.G4 U1.G4
TEMP_CH0: C8.1 Q1.2 TP25.1 U0.F3
TEMP_CH1: C17.1 Q2.2 TP28.1 U0.F2
TEMP_CH2: C33.1 Q3.2 TP31.1 U1.F3
TEMP_CH3: C44.1 Q4.2 TP34.1 U1.F2
UNUSED1: J3.9 J4.9
UNUSED2: J3.10 J4.10
USB_3.3V: J2.5 M6.3 M7.3
USB_5V: C60.1 C61.1 J2.1 J3.8 J4.8 R59.2 R60.2 U10.4
VDD33_A: C30.1 C58.1 C64.1 JP1.1 LED8.A LED9.A M6.2 R52.1 R53.1 R55.1 R56.1 R57.1 R58.1 R63.2 R64.2 R67.2 R68.2 R71.2 R72.2 R75.2 R76.2 R80.1 RPU2.R1_2 RPU2.R2_2 RPU2.R3_2 RPU2.R4_2 RPU3.R1_2 RPU3.R2_2 RPU3.R3_2 RPU3.R4_2 SW2.SW1 U0.D2 U0.E2 U8.8 U9.18 U11.1 U11.3 U12.5
VDD33_B: C55.1 M7.2 R41.2 R65.2 R66.2 R69.2 R70.2 R73.2 R74.2 R77.2 R78.2 R81.2 U1.D2 U1.E2
VDDIO: JP1.2 M9.1 M10.1 R26.2 R27.2 R49.2 R50.2 R51.1 RPU1.R1_2 RPU1.R2_2 RPU1.R3_2 RPU1.R4_2 U0.C7 U1.C7
VFB0: R10.1 R11.1 R12.1 U3.10
VFB1: R19.1 R20.2 R21.1 U4.6
VFB2: C37.2 R31.1 R32.1 R33.2 U6.11
VFB3: R42.2 R44.2 R45.1 U7.2
VOUT_CH0 [HV]: C13.+ NB21.2 R12.2 R17.2 RL0.2 RSNS2.2 TP0.TP
VOUT_CH1 [HV]: C21.+ NB4.1 R21.2 R24.2 RL1.2 RSNS3.2 TP1.TP
VOUT_CH2: C39.+ NB2.1 R33.1 R35.2 R38.2 RL2.2 RSNS4.2 TP2.TP
VOUT_CH3: C50.- NB7.1 R45.2 R48.2 RL3.2 RSNS5.2 TP3.TP
VOUT_SNS_CH0 [HV]: C14.1 R17.1 U0.A2
VOUT_SNS_CH1 [HV]: C23.1 R24.1 U0.A6
VOUT_SNS_CH2: C41.1 R38.1 U1.A2
VOUT_SNS_CH3: C52.1 R48.1 U1.A6
VP5P0: C26.1 C27.2 C53.1 L4.2 U0.G2 U1.G2 U5.4
VP48V_U0 [HV]: C7.1 C16.1 NB13.1 RSNS0.2 U0.G1 U3.30 U3.31 U3.32 U4.4
VP48V_U1 [HV]: C32.1 C42.1 C43.1 L6.1 NB18.1 RSNS1.2 U1.G1 U6.1 U7.10

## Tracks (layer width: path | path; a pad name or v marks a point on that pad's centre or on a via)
+12V  (via drill 0.25)
  Top 0.152: R1.2 92.2,53.09 91.69,53.59 v91.69,56.01
  Route2 0.203: v88.39,46.23 88.39,51.05 88.65,51.31 v88.65,56.39
  Bottom 0.152: R79.2 116.62,56.43 115.82,55.63 115.57,55.63 | 115.57,55.63 TP14.TP | U2.27 87.26,45.72 | 115.57,55.63 arc-35 114.94,56.13 114.94,55.88 | 114.94,55.88 114.94,55.37 | 114.94,55.37 114.94,55.12 arc-35 115.57,55.63 | 115.57,55.63 arc-35 114.94,55.88 | 114.94,55.37 arc-35 115.57,55.63
  Bottom 0.203: 87.26,45.72 87.88,45.72 v88.39,46.23 | v88.65,56.39 87.68,56.39 C2.1
  pour Bottom (no thermals): 92.2,59.69 95.76,59.69 97.03,58.67 105.66,58.67 112.52,65.28 115.32,65.28 116.59,64.01 116.59,61.98 115.06,60.45 112.27,60.45 107.57,55.75 85.34,55.75 85.34,56.9 87.88,56.9
  pour Route2 (no thermals): 116.59,45.21 115.57,46.23 115.57,57.91 111.76,61.72 111.76,64.26 113.03,65.28 115.06,65.28 116.84,63.5 116.84,47.24 118.11,45.97 118.11,24.89 111.25,18.03 111.25,1.02 111,0.76 110.24,0.76 109.98,1.02 109.98,19.05 116.59,25.65
  pour Top (no thermals): 115.32,60.71 115.32,49.28 112.78,49.28 112.78,53.34 111.25,54.86 111.25,56.39 112.01,57.15 112.01,61.21 111.51,61.72 111.51,64.01 111.76,64.26 111.76,73.41 109.98,75.18 109.98,78.23 110.24,78.49 111,78.49 111.51,77.98 111.51,74.93 113.03,73.41 113.03,67.56 116.59,64.01 116.59,61.98
+48V  (via drill 0.25)
  Route2 0.152: v84.2,35.56 84.2,38.48 v85.09,39.37
  Route15 0.152: v109.22,45.21 97.66,45.21 94.87,42.42 | 94.87,42.42 TP15.TP | 94.87,42.42 arc-35 93.85,42.04 93.98,41.91 | 93.98,41.91 94.36,41.53 | 94.36,41.53 94.49,41.4 arc-35 94.87,42.42 | 94.87,42.42 arc-35 93.98,41.91 | 94.36,41.53 arc-35 94.87,42.42
  Bottom 0.152: RSNS0.1 75.18,48.51 74.93,48.26 NB12.1 | R28.1 v109.22,45.21 | U5.1 84.29,34.76 84.33,34.8 84.2,34.8 v84.2,35.56 | R6.2 v85.09,39.37 | v85.09,39.37 90.68,39.37 | 90.68,39.37 90.93,39.37 | 90.93,39.37 91.19,39.37 | 91.19,39.37 91.82,39.37 TP15.TP | v85.09,39.37 82.8,39.37 82.04,38.61 C24.1 | 90.68,39.37 arc35 91.57,39.88 92.33,38.99 arc20 90.68,39.37 | 90.93,39.37 arc35 91.82,39.88 | 91.19,39.37 arc35 92.08,39.88
  Bottom 0.203: NB17.1 74.93,39.88 75.18,39.62 RSNS1.1
  Bottom 0.254: C24.1 81.79,37.08 81.4,36.7 U5.8
  pour Bottom (no thermals): 78.49,56.13 80.01,56.13 80.9,57.02 84.33,57.02 84.33,55.75 81.66,55.75 79.88,53.85 78.49,53.85 76.71,52.07 76.71,40.13 76.96,40.13 79.25,37.59 82.55,37.59 82.55,36.32 78.99,36.32 76.71,38.86 75.69,38.86 75.69,52.2 78.49,54.99
+48V_EN  (via drill 0.25)
  Top 0.152: TP36.1 92.96,48.51 92.2,49.28 R1.1 R2.2
  Route2 0.152: v89.41,46.23 90.17,46.23 90.68,46.74 TP36.1
  Bottom 0.152: U2.25 87.25,46.74 87.88,46.74 88.14,46.99 88.65,46.99 v89.41,46.23
A0_MUX  (via drill 0.25)
  Top 0.152: U9.3 100.71,13.46 v100.46,13.21 100.2,13.34 99.29,13.34 RPU3.R2_1
  Bottom 0.152: JP2.6 100.46,12.83 v100.46,13.21
A1_MUX  (via drill 0.25)
  Top 0.152: U9.2 100.85,13.96 100.71,14.1 v100.46,14.1 99.29,14.1 RPU3.R3_1
  Bottom 0.152: JP2.7 v100.46,14.1
A2_MUX  (via drill 0.25)
  Top 0.152: U9.1 101.11,14.46 101.03,14.54 v100.46,14.99 99.3,14.99 RPU3.R4_1
  Bottom 0.152: 99.27,15.54 99.44,15.62 100.2,15.62 100.46,15.49 v100.46,14.99
  Bottom 0.254: 99.27,15.54 99.27,15.38 JP2.8
ALERTB  (via drill 0.25)
  Top 0.152: U0.E5 v57.67,57.91 | v57.67,23.62 U1.E5
  Route2 0.152: v57.67,57.91 57.67,57.06 57.02,56.39 57.02,55.5 57.28,55.24 57.28,54.36 57.02,54.1 57.02,33.66 v56.9,33.27 57.15,33.02 57.15,29.46 56.52,28.83 56.52,27.94 57.15,27.3 57.15,24.13 v57.67,23.62 | v28.45,38.48 v28.45,33.78
  Route15 0.152: v13.72,33.27 14.22,33.78 v28.45,33.78 55.88,33.78 56.39,33.27 v56.9,33.27
  Bottom 0.152: 12.45,38.1 12.45,37.85 11.5,36.9 M10.2 11.35,36.07 10.16,36.07 9.27,35.18 9.27,34.42 10.03,33.66 13.34,33.66 v13.72,33.27 16.36,30.63 RPU1.R3_1 | 12.45,38.1 TP6.TP | v28.45,38.48 28.59,38.62 U12.1 | 12.45,38.1 arc-35 12.95,38.99 12.7,38.99 | 12.7,38.99 12.19,38.99 | 12.19,38.99 11.94,38.99 arc-35 12.45,38.1 | 12.19,38.99 arc-35 12.45,38.1 | 12.45,38.1 arc-35 12.7,38.99
ALERTB_3V3  (via drill 0.25)
  Route2 0.152: J3.3 100.65,74.48 97.92,71.75 97.92,68.96 99.31,67.56 99.31,52.07 99.44,51.94 v99.44,38.1 v99.44,29.97 99.44,5.71 100.58,4.57 100.58,3.6 J4.3 | v16,35.56 v16,37.85
  Route15 0.152: J2.6 121.28,38.1 v99.44,38.1 69.6,38.1 68.58,39.12 60.71,39.12 60.2,38.61 52.07,38.61 51.56,39.12 34.54,39.12 33.27,37.85 v16,37.85
  Bottom 0.152: R53.2 v99.44,29.97 99.39,29.97 | M10.3 v16,35.56
CTRL  (via drill 0.25)
  Top 0.152: U1.E7 U1.D7 60.4,23.88 v61.72,23.88 | U0.D7 U0.E7 60.17,57.4 v61.47,57.4 | v110.24,25.4 111.48,25.4 S1.2 S1.5
  Route2 0.152: J4.2 98.65,1.55 97.54,2.67 97.54,4.83 98.3,5.59 v98.3,25.4 98.3,31.88 98.17,32 v98.17,47.75 98.17,67.44 96.9,68.71 96.9,75.95 98.68,77.72 J3.2 | v61.47,57.4 v61.47,47.75 63.25,46.1 63.25,34.04 62.48,33.27 62.48,27.18 61.72,26.42 v61.72,23.88
  Route15 0.152: v110.24,25.4 v98.3,25.4 | v61.47,47.75 v98.17,47.75
  Bottom 0.152: RPU2.R1_1 95.25,71.95 95.25,72.64 94.23,73.66 94.23,76.71 94.49,76.96 | 94.49,76.96 94.53,77 R54.2 95.54,76.96 | 95.54,76.96 96.52,76.96 97.54,77.72 J3.2 | 94.49,76.96 95.54,76.96 | C57.1 v110.24,25.4
CTRL_P  (via drill 0.25)
  Route15 0.152: v95.25,73.91 103.89,73.91 105.79,72.01 | 105.79,72.01 106.17,71.63 | 106.17,71.63 TP13.TP | 105.79,72.01 arc35 107.06,71.5 106.93,71.37 | 106.93,71.37 106.43,70.87 | 106.43,70.87 106.3,70.74 arc35 105.79,72.01 | 106.17,71.63 arc35 106.93,71.37 | 106.43,70.87 arc35 106.17,71.63
  Bottom 0.152: R54.1 v95.25,73.91
DAC_CH0  (via drill 0.25)
  Top 0.152: U0.B2 54.63,60.91 54.63,61.8 54.36,62.1 v54.36,62.74 | R10.2 v78.23,45.72
  Route2 0.152: v68.83,46.86 68.83,48.26 67.31,49.78 67.31,54.36 67.56,54.61 TP26.1 v67.56,64.52 | v54.36,64.52 v54.36,62.74
  Route15 0.152: v78.23,45.72 72.39,45.72 71.25,46.86 v68.83,46.86 | v67.56,64.52 v54.36,64.52
DAC_CH1  (via drill 0.25)
  Top 0.152: TP29.1 43.69,59.47 R19.2 | U0.B4 57.15,60.45 v56.66,60.9
  Route15 0.152: v56.66,60.9 56.21,60.88 56.01,61.09 53.09,61.09 52.96,61.21 52.2,61.21 52.07,61.09 47.37,61.09 45.97,62.48 44.45,62.48 TP29.1
DAC_CH2  (via drill 0.25)
  Top 0.152: TP32.1 R31.2 | U1.B2 v54.66,26.62
  Route15 0.152: v54.66,26.62 53.85,27.43 25.4,27.43 TP32.1
DAC_CH3  (via drill 0.25)
  Top 0.152: U1.B4 57.15,26.16 v57.67,26.63 | v84.84,9.78 R42.1 84.8,10.92 83.82,10.92 83.82,12.45 83.78,12.48 R41.1
  Route2 0.152: v67.82,10.16 66.29,11.68 66.29,28.45 TP35.1
  Route15 0.152: v57.67,26.63 62.05,26.62 62.23,26.8 62.74,26.8 62.92,26.62 65.48,26.62 66.04,27.05 TP35.1 | v84.84,9.78 74.3,9.78 73.91,10.16 v67.82,10.16
EESCL  (via drill 0.25)
  Route2 0.152: v112.78,18.03 120.14,25.4 120.14,32.96 J2.11
  Bottom 0.152: U10.1 111.69,9.21 111,9.91 111,14.73 111.76,15.49 111.76,17.02 R60.1 112.74,18 v112.78,18.03
EESDA  (via drill 0.25)
  Route2 0.152: v112.78,16 122.17,25.4 122.17,32.99 J2.12
  Bottom 0.152: U10.3 111.83,11.11 111.51,11.43 111.51,14.48 112.01,14.99 R59.1 112.74,15.96 v112.78,16
FAULTB  (via drill 0.25)
  Top 0.152: U1.G7 U1.F6 60.2,21.08 v60.96,21.08 | v60.71,54.86 U0.G7 U0.F6
  Route2 0.152: v60.96,21.08 60.96,21.21 60.71,21.46 60.71,23.62 60.45,23.88 60.45,29.08 59.69,29.84 v59.69,39.37 59.69,45.97 60.71,46.99 v60.71,54.86 | v18.54,32.77 v18.54,38.48 18.54,44.7 14.35,48.9 | 14.35,48.9 14.22,49.02 | 14.22,49.02 TP5.TP | 14.35,48.9 arc-35 13.84,50.04 13.72,49.91 | 13.72,49.91 13.34,49.53 | 13.34,49.53 13.21,49.4 arc-35 14.35,48.9 | 13.34,49.53 arc-35 14.22,49.02 | 14.22,49.02 arc-35 13.72,49.91
  Route15 0.152: v18.54,38.48 v26.67,38.48 27.3,38.48 27.94,39.12 28.96,39.12 29.21,38.86 33.53,38.86 34.54,39.88 51.82,39.88 52.32,39.37 v59.69,39.37
  Bottom 0.152: M9.2 11.5,47.06 12.45,48.01 12.45,48.39 | 12.45,48.39 TP5.TP | RPU1.R4_1 18.58,32.73 v18.54,32.77 | v26.67,38.48 26.67,39.37 26.84,39.54 U12.3 | 12.45,48.39 arc-35 12.95,49.02 12.7,49.02 | 12.7,49.02 12.19,49.02 | 12.19,49.02 11.94,49.02 arc-35 12.45,48.39 | 12.19,49.02 arc-35 12.45,48.39 | 12.45,48.39 arc-35 12.7,49.02
FAULTB_3V3  (via drill 0.25)
  Route2 0.152: J3.1 98.65,74.52 97.41,73.28 97.41,68.83 98.81,67.44 v98.81,32.26 98.81,25.78 98.93,25.65 98.93,25.15 98.81,25.02 98.81,4.95 98.65,4.83 J4.1 | J4.1 | J4.1 | v19.56,3.56 9.65,13.46 9.65,33.27 9.14,33.78 v9.14,44.96
  Route15 0.152: v19.56,3.56 98.03,3.56 J4.1
  Bottom 0.152: R52.2 v98.81,32.26 | v9.14,44.96 10.16,43.94 12.7,43.94 13.46,44.7 13.46,45.65 M9.3
GND  (via drill 0.25)
  Top 0.152: U0.C2 U0.C3 | U0.C3 U0.B3 | U0.C3 U0.D4 | U0.D4 U0.D5 U0.D6 U0.C6 U0.B5 U0.A5 | U0.F4 U0.E4 U0.D4 | U1.C2 U1.C3 | U1.C3 U1.B3 | U1.C3 U1.D4 | U1.B5 U1.C6 | U1.C6 U1.D5 U1.D4 | U1.F4 U1.E4 U1.D4 | U1.C6 59.15,25.16 v59.65,25.63 | U9.17 104.64,13.96 U9.PAD
  other vias: 22.35,17.14 23.37,17.14 25.4,17.14 26.42,17.14 34.54,17.14 36.07,17.14 61.47,42.42 61.47,39.88 52.83,42.42 102.36,63.75 102.36,61.72 102.36,59.69 102.36,47.5 102.36,44.45 104.14,32.26 104.14,29.72 104.14,13.46 52.32,62.74 105.16,67.56 58.17,62.74 64.52,54.86 68.07,21.72 84.07,17.91 84.07,17.14 85.09,17.14 85.09,17.91 52.83,40.13 54.36,13.46 59.94,13.46 57.15,13.46 104.14,27.18 102.36,67.56 54.99,53.98 102.36,55.24 102.36,52.7 102.36,50.16 111,32.26 111,34.8 111,29.72 47.5,57.66 55.65,59.92 58.66,57.91 56.64,26.63
  pour Route2 (rank 2, no thermals): 0.76,0.25 0.25,0.76 0.25,80.52 0.76,81.03 123.7,81.03 124.21,80.52 124.21,0.76 123.7,0.25
  pour Route15 (rank 2, no thermals): 1.02,0.25 0.25,1.02 0.25,80.26 1.02,81.03 123.44,81.03 124.21,80.26 124.21,1.02 123.44,0.25
  pour Bottom (rank 2, no thermals): 1.27,0.25 0.25,1.27 0.25,80.01 1.27,81.03 123.19,81.03 124.21,80.01 124.21,1.27 123.19,0.25
  pour Top (rank 2, no thermals): 0.25,80.77 0.51,81.03 123.95,81.03 124.21,80.77 124.21,0.51 123.95,0.25 0.51,0.25 0.25,0.51
  pour Bottom (no thermals): 83.44,50.16 81.79,51.82 81.79,53.98 87.88,53.98 87.88,51.82 86.23,50.16
IIN_SNSM0  (via drill 0.25)
  Top 0.152: U0.E1 53.36,57.42 v53.34,57.4
  Route2 0.152: v53.34,57.4 52.45,56.52 v52.45,53.47 | v70.36,52.7 v70.36,45.97
  Route15 0.152: v52.45,53.47 52.96,52.96 63.75,52.96 64.01,52.7 v70.36,52.7
  Bottom 0.152: v70.36,45.97 73.91,45.97 74.42,46.48 NB13.2
IIN_SNSM1  (via drill 0.25)
  Top 0.152: U1.E1 53.32,23.13 v53.21,23.24
  Route2 0.152: v53.21,23.24 53.21,23.75 53.34,23.88 53.34,25.65 52.58,26.42 52.58,32 55.12,34.54 v55.12,40.89
  Route15 0.152: v55.12,40.89 71.37,40.89 72.14,41.66 v74.17,41.66
  Bottom 0.152: NB18.2 74.42,41.4 v74.17,41.66
IIN_SNSP0  (via drill 0.25)
  Top 0.152: U0.F1 53.61,55.88 v53.34,55.88
  Route2 0.152: v53.34,55.88 v53.34,53.98 | v71.12,53.09 v71.12,45.34
  Route15 0.152: v53.34,53.98 53.98,53.34 64.01,53.34 64.26,53.09 69.85,53.09 70.1,53.34 70.87,53.34 v71.12,53.09
  Bottom 0.152: v71.12,45.34 74.04,45.34 74.93,46.23 NB12.2
IIN_SNSP1  (via drill 0.25)
  Top 0.152: U1.F1 53.31,22.13 v53.21,22.23
  Route2 0.152: v53.21,22.23 52.45,22.99 52.45,23.62 52.83,24 52.83,25.4 52.07,26.16 52.07,32.26 54.74,34.92 54.74,39.88 54.36,40.26 v54.36,41.66
  Route15 0.152: v54.36,41.66 55.37,41.66 55.75,41.27 71.12,41.27 72.14,42.29 v74.68,42.29
  Bottom 0.203: v74.68,42.29 74.93,42.04 NB17.2
INTVCC
  Top 0.152: U3.9 82.04,50.97 82.04,51.44 82.42,51.69 | 82.42,51.69 82.42,54.74 82.04,55.12 81.53,55.12 81.51,55.14 U3.21 81.53,56.13 81.53,56.64 81.41,56.9 81.41,57.91 81.79,58.29 84.84,58.29 85.72,57.4 85.72,56.48 C11.1 | 82.42,51.69 82.68,51.56 83.26,51.56 U3.11 83.37,51 84.33,50.04 R9.1 84.37,48.51 85.09,48.51 85.34,48.26 85.34,47.24 85.64,46.95 R82.1
IOUT_SNSM_CH0  (via drill 0.25)
  Top 0.152: U0.A3 56.15,63.23 56.13,63.25 v56.13,66.29 | v86.61,62.23 89.41,62.23 | R14.2 89.95,61.68 89.41,62.23 | 89.41,62.23 89.92,62.74 89.92,63.72 R16.2 89.92,63.79 89.92,64.52 89.66,64.77 88.65,64.77 88.35,65.06 C15.2
  Route15 0.152: v56.13,66.29 57.66,66.29 58.29,65.66 75.82,65.66 77.47,64.01 85.85,64.01 86.61,63.25 v86.61,62.23
IOUT_SNSM_CH1  (via drill 0.25)
  Top 0.152: U0.A7 60.15,62.69 v60.2,62.74
  Route15 0.152: v60.2,62.74 59.56,62.1 48.26,62.1 46.35,64.01 40.89,64.01 v40.13,64.77
  Bottom 0.152: R23.1 39.03,64.77 C22.2 39.03,64.68 39.12,64.77 v40.13,64.77
IOUT_SNSM_CH2  (via drill 0.25)
  Top 0.152: v56.13,29.84 56.13,27.15 U1.A3
  Route2 0.152: v46.99,22.1 46.99,28.83 46.35,29.46 v46.35,29.84
  Route15 0.152: v46.35,29.84 v56.13,29.84
  Bottom 0.152: 47.5,20.79 C40.2 | C40.2 47.54,21.55 v46.99,22.1 | R37.2 47.5,19.09 47.5,20.57 47.62,20.74 C40.2
IOUT_SNSM_CH3  (via drill 0.25)
  Top 0.152: U1.A7 60.2,27.18 v63.75,27.18
  Route2 0.152: v63.75,27.18 63.75,26.16 62.87,25.27 62.87,17.02 63.12,16.76 v63.12,16.26
  Bottom 0.152: R46.1 64.9,15.24 64.77,15.11 63.15,15.11 C51.1 v63.12,16.26
IOUT_SNSP_CH0  (via drill 0.25)
  Top 0.152: U0.A4 v57.15,65.66 | v86.61,59.94 89.92,59.94 | 89.92,59.94 90.68,59.94 91.19,60.45 91.19,65.53 90.93,65.79 C15.1 R15.2 | R13.2 89.95,58.97 89.92,59.05 89.92,59.94
  Route15 0.152: v57.15,65.66 57.66,65.66 58.04,65.28 75.69,65.28 77.47,63.5 84.84,63.5 85.72,62.61 85.72,60.83 v86.61,59.94
IOUT_SNSP_CH1  (via drill 0.25)
  Top 0.152: U0.B7 60.17,60.42 v61.21,61.47
  Route15 0.152: v61.21,61.47 60.71,61.47 60.45,61.72 48.01,61.72 46.1,63.63 v40.13,63.63
  Bottom 0.152: R22.1 39.03,62.99 C22.1 39.03,63.08 39.12,62.99 39.88,62.99 40.13,63.25 v40.13,63.63
IOUT_SNSP_CH2  (via drill 0.25)
  Top 0.152: v57.15,28.45 U1.A4
  Route2 0.152: v46.35,22.61 v46.35,28.7
  Route15 0.152: v46.35,28.7 54.1,28.7 54.36,28.45 v57.15,28.45
  Bottom 0.152: 45.97,20.79 C40.1 | C40.1 45.94,22.19 v46.35,22.61 | R36.2 45.97,19.09 45.97,20.57 45.85,20.74 C40.1
IOUT_SNSP_CH3  (via drill 0.25)
  Top 0.152: v62.48,26.16 60.18,26.16 U1.B7
  Route2 0.152: v62.1,14.48 62.1,14.99 62.48,15.37 v62.48,26.16
  Bottom 0.152: R47.1 64.9,13.72 64.77,13.84 63.15,13.84 C51.2 62.99,13.72 62.87,13.84 62.1,13.84 v62.1,14.48
N$1  (via drill 0.25)
  Route15 0.152: v32.26,43.43 31.62,42.8 v28.7,42.8
  Bottom 0.152: R61.1 v32.26,43.43 | v28.7,42.8 28.7,41.85 U12.6
N$2  (via drill 0.25)
  Top 0.203: SW2.SW2 v21.34,36.58
  Route2 0.203: v21.34,36.58 21.34,25.4 21.08,25.15 21.08,24.13 21.34,23.88 v21.34,9.14
  Bottom 0.152: M8.1 22.57,9 R34.1 22.57,9.11 22.61,9.14 v21.34,9.14
N$3  (via drill 0.25)
  Top 0.152: v32.26,39.62 31.75,39.24 LED8.C
  Bottom 0.152: R61.2 v32.26,39.62
N$4
  Top 0.152: U3.16 83.96,54.09 84.2,54.1 R7.2
N$5  (via drill 0.25)
  Top 0.152: LED4.C v40.89,9.14
  Bottom 0.152: v40.89,9.14 39.62,9.14 39.37,8.89 M3.3
N$6  (via drill 0.25)
  Top 0.152: LED2.C 73.41,71.12 v73.91,70.61
  Bottom 0.152: v73.91,70.61 75.18,70.61 75.44,70.87 M1.3
N$7
  Top 0.152: LED2.A 73.42,73.15 73.91,73.15 74.17,72.9 74.17,72.39 74.93,72.39 74.93,71.97 R67.1
N$8
  Bottom 0.152: 87.27,45.21 U2.28 87.38,45.21 87.38,44.7 87.88,44.2 C4.1
N$9
  Top 0.152: LED4.A 39.14,6.33 R69.1
N$10  (via drill 0.25)
  Top 0.152: LED3.C 40.28,71.61 40.13,71.5 v40.13,70.61
  Bottom 0.152: v40.13,70.61 38.35,70.61 38.1,70.87 M2.3
N$11
  Top 0.152: LED3.A 40.88,73.15 40.26,73.15 40.13,73.03 40.13,72.52 40.01,72.39 39.5,72.39 39.37,72.26 39.37,71.88 39.12,71.88 R68.1
N$12  (via drill 0.25)
  Top 0.152: LED1.A 118.73,54.85 v118.75,54.86
  Bottom 0.152: v118.75,54.86 117.64,54.86 R79.1
N$13
  Bottom 0.152: U2.3 81.41,46.25 81.41,47.75 82.44,47.75 U2.6
N$14  (via drill 0.25)
  Top 0.152: U1.C5 v57.66,25.62 v57.67,25.62 | v51.18,25.65 51.18,26.63 C54.1
  Route15 0.152: v57.67,25.62 56.85,25.62 56.82,25.65 52.45,25.65 52.35,25.75 51.35,25.75 v51.18,25.65
N$15  (via drill 0.25)
  Top 0.152: U1.C4 57.17,25.13 v57.67,24.64 | v49.4,25.65 49.4,26.63 C54.2
  Route15 0.152: v57.67,24.64 52.45,24.64 52.32,24.51 50.55,24.51 v49.4,25.65
N$16
  Top 0.152: R70.1 73.43,6.31 LED5.A
N$17  (via drill 0.25)
  Top 0.152: LED5.C v73.41,9.14
  Bottom 0.152: v73.41,9.14 74.68,9.14 74.93,8.89 M4.3
N$18
  Bottom 0.152: R3.2 88.52,43.05 88.01,43.05 86.61,44.45 86.23,44.45 U2.30
N$19
  Top 0.152: C56.1 51.4,24.64 51.44,24.64 51.56,24.51 52.32,24.51 52.45,24.64 55.65,24.64 U1.D3 56.15,23.96 56.19,23.93 56.19,23.33 56.15,23.29 U1.E3
N$20
  Top 0.152: U3.8 81.53,50.84 81.53,50.04 81.28,49.78 76.45,49.78 76.2,49.53 R8.2
N$21
  Bottom 0.152: U2.32 85.09,43.68 84.33,42.93 83.69,42.93 83.57,42.8 C5.1
N$22
  Top 0.203: U7.6 85.58,20.72 84.96,21.34 84.96,22.12 M5.3 M5.2 M5.1
  Top 0.254: R43.2 78.49,21.08 79.5,22.1 83.53,22.1 M5.1
N$23  (via drill 0.25)
  Route2 0.152: v80.77,31.75 82.04,30.48 v83.31,30.48
  Bottom 0.152: U5.5 80.81,32.81 80.77,32.77 v80.77,31.75 | v83.31,30.48 83.82,30.48 84.33,29.97 C25.1
N$24
  Bottom 0.152: U11.4 27.62,68.17 C62.2
N$25  (via drill 0.25)
  Bottom 0.152: R62.2 v30.23,43.43 27.81,43.43 27.3,42.93 27.3,41.76 U12.4
N$26  (via drill 0.25)
  Top 0.152: LED9.C 29.72,39.24 v30.23,39.62
  Bottom 0.152: v30.23,39.62 R62.1
N$27  (via drill 0.25)
  Top 0.152: NB1.1 44.45,16 44.2,16.26 RSNS4.1 | C37.1 31.76,22.35
  Top 0.254: U6.12 31.76,22.35 31.76,21.86 v31.75,21.84 | v41.91,21.08 43.71,21.08 C38.1
  Route15 0.254: v31.75,21.84 35.31,21.84 36.07,21.08 v41.91,21.08
  pour Top (no thermals): 42.93,21.21 45.47,21.21 45.47,19.94 44.96,19.43 44.96,16.64 43.31,16.64 43.31,19.56 42.93,19.94
N$28
  Top 0.152: M12.5 M12.6 47.64,43.29 48.13,42.8 49.66,42.8 50.16,43.31 50.16,44.08 LED11.2
N$30
  pour Bottom (no thermals): 92.2,51.56 92.2,50.29 91.44,49.53 83.31,49.53 83.06,49.28 81.79,49.28 81.03,50.04 81.03,51.31 80.26,52.07 78.49,52.07 77.47,50.8 79.25,49.78 80.52,48.64 82.68,48.64 83.31,48.01 86.36,48.01 86.87,48.51 91.44,48.51 92.2,47.75 92.2,47.5 94.61,48.51 95.63,51.56
N$32
  Bottom 0.152: U2.33 84.59,43.95 83.95,43.31 82.17,43.31 81.79,42.93 81.79,42.42 82.04,42.16 82.04,42.2 R4.2
N$33
  Top 0.152: R18.2 35.69,60.67 35.69,59.69 36.32,59.05 U4.8
N$34
  Top 0.152: M5.4 85.6,22.13 85.6,21.34 86.11,20.83 86.11,18.92 85.98,18.8 85.22,18.8 85.09,18.92 85.09,19.67 U7.7
N$35
  Top 0.203: U6.18 35.66,24.48 35.81,24.64 36.32,24.64 37.34,25.65 C36.1
N$36  (via drill 0.25)
  Top 0.152: NB3.1 33.78,67.82 33.53,68.07 RSNS3.1 | U4.1 35.32,53.32 35.23,53.47 v34.62,53.47 | v30.61,62.99 30.61,63.88 30.71,63.98 C20.1
  Route2 0.152: v34.62,53.47 30.61,57.4 v30.61,62.99
  pour Top (no thermals): 22.73,59.44 25.02,59.44 25.02,59.69 28.7,63.37 33.66,63.37 33.66,64.64 33.02,65.41 33.02,68.83 31.88,68.83 31.88,65.28 31.24,64.64 27.43,64.64 22.73,59.94
N$37  (via drill 0.25)
  Top 0.152: U6.16 34.36,21.15 v34.29,21.08 | v29.72,20.32 C34.1
  Route15 0.152: v34.29,21.08 31.75,21.08 30.99,20.32 v29.72,20.32
N$38
  Top 0.152: R30.1 32.51,30.48 32.38,30.35 32.38,29.29 U6.8
N$39
  pour Top (no thermals): 36.83,15.88 38.86,15.88 40.51,17.4 40.51,24 36.83,24 36.83,23.11 38.99,23.11 39.37,22.73 39.37,18.41 38.73,17.65 36.83,17.65
N$40
  pour Top (no thermals): 32.92,24.13 33.2,24.13 33.2,22.73 33.27,22.61 33.27,19.94 33.78,18.29 33.78,15.88 31.75,15.88 31.75,17.65 32.77,20.19 32.77,22.61 32.92,22.78
N$41
  Top 0.203: U6.10 31.11,30.1 30.48,30.73 C35.1
N$42
  Top 0.152: U7.3 84.58,14.73 84.84,14.48 86.23,14.48 87.12,15.37 88.43,15.37 C46.1
N$43
  pour Top (no thermals): 85.72,23.24 85.72,25.78 84.58,26.92 79.76,26.92 79.38,26.54 74.42,26.54 74.42,25.65 82.8,25.65 83.44,25.02 83.44,23.24
N$44
  pour Top (no thermals): 81.53,24.13 79.76,24.13 79.25,24.64 74.42,24.64 74.42,23.62 74.8,23.24 74.8,17.27 76.33,17.27 76.33,23.62 78.99,23.62 79.76,22.86 81.53,22.86
N$45
  Top 0.152: U7.4 85.08,16.12 85.22,16.26 86.23,16.26 87.38,17.4 88.48,17.4 R40.2
N$46
  pour Bottom (no thermals): 76.2,35.05 79.38,35.05 80.26,34.29 81.66,34.29 81.66,33.99 80.26,33.99 79.88,33.86 76.2,33.86
N$47
  Top 0.152: R39.2 80.77,13.72 82.04,14.99 83.57,14.99 83.57,15.36 U7.1
N$48
  Bottom 0.152: R25.1 86.07,33.78 85.34,33.78 85.02,33.46 U5.3
N$49  (via drill 0.25)
  Top 0.152: U0.C4 57.17,59.42 v57.65,58.93 | v49.66,59.31 49.66,60.11 C29.2
  Route15 0.152: v57.65,58.93 56.81,58.91 56.62,58.8 54.36,58.8 53.98,58.42 50.55,58.42 v49.66,59.31
N$50
  Top 0.152: C45.1 R39.1
N$51
  Bottom 0.152: R5.2 R6.1 85.08,42.01 85.08,42.91 85.6,43.43 U2.31
N$52
  Top 0.152: U0.E3 U0.D3 56.13,58.42 55.63,58.93 53.09,58.93 52.32,58.17 C31.2
N$53  (via drill 0.25)
  Top 0.152: U0.C5 58.15,59.45 v57.65,59.93 | v51.31,59.31 51.31,60.16 C29.1
  Route15 0.152: v57.65,59.93 57.15,59.94 56.52,59.31 53.72,59.31 53.21,58.8 51.69,58.8 v51.31,59.31
N$54
  Bottom 0.152: C62.1 25.72,68.17 U11.5 23.38,70.02 C63.1 22.52,70.02 21.84,69.34 21.23,69.34 | 21.23,69.34 20.35,69.34 JP1.3 | 21.23,69.34 arc-35 20.78,69.6 20.78,69.14 arc-35 21.23,69.34
N$55
  Bottom 0.406: M8.3 R35.1
N$56  (via drill 0.25)
  Top 0.152: v50.16,46.99 50.16,45.84 LED11.1
  Route2 0.152: v48.51,43.43 50.16,45.09 v50.16,46.99
  Bottom 0.152: R72.1 48.48,44.36 48.51,44.32 v48.51,43.43
N$57
  Top 0.152: LED11.4 49.11,44.11 48.26,44.96 46.99,44.96 46.48,45.47 46.48,45.99 M12.3
N$58  (via drill 0.25)
  Top 0.152: LED10.1 64.87,46.83 v64.9,46.99
  Route2 0.152: v64.9,46.99 64.9,44.32 v65.79,43.43
  Bottom 0.152: v65.79,43.43 R71.1
N$59
  Top 0.152: C18.1 37.08,60.74 37.08,59.69 36.82,59.43 U4.7
N$60  (via drill 0.25)
  Top 0.152: LED10.3 64.17,46.58 v63.88,46.99
  Route2 0.152: v63.88,46.99 63.88,44.2 65.53,42.55 v67.31,42.55
  Bottom 0.152: v67.31,42.55 R75.1
N$61
  Bottom 0.152: C3.1 R3.1
N$62
  Top 0.152: NB6.1 69.34,14.73 69.6,14.99 RSNS5.1
  pour Top (no thermals): 70.36,15.37 70.36,16.64 70.23,17.53 70.23,22.61 70.74,23.11 70.74,24.64 68.58,24.64 68.58,22.99 68.96,22.61 68.96,17.14 68.83,16.76 68.83,15.37
N$63  (via drill 0.25 pad 0.25)
  Top 0.152: v64.52,57.4 62.74,57.4 LED6.A
  Bottom 0.152: R80.2 63.75,57.37 63.75,57.4 v64.52,57.4
N$64
  Top 0.152: C8.2 64.94,50.51 63.63,51.82 63.63,54.74 62.99,55.37 62.99,56.11 NB5.2
  pour Top (no thermals): 73.15,52.32 73.91,52.32 73.91,51.31 73.28,50.67 73.28,49.91 72.52,49.91 72.01,50.42 68.83,50.42 68.83,50.93 72.52,50.93 73.15,51.56
N$65  (via drill 0.25 pad 0.25)
  Top 0.152: v64.52,23.62 62.74,23.62 LED7.A
  Bottom 0.152: R81.1 63.5,23.62 v64.52,23.62
N$66
  Top 0.152: U9.4 101.1,12.96 100.58,12.45 100.58,9.61 R58.2 C59.1
N$67
  Top 0.152: NB14.2 45.72,57.66 44.96,56.9 43.98,56.9 C17.2
  pour Top (no thermals): 40.51,54.99 41.02,54.99 41.02,55.63 41.91,56.52 44.45,56.52 44.45,57.28 41.15,57.28 40.51,56.64
N$68  (via drill 0.25)
  Top 0.152: v51.31,28.07 52.43,28.07 NB15.2 | v43.18,30.23 42.93,29.97 41.95,29.97 C33.2
  Route15 0.152: v43.18,30.23 44.96,30.23 45.72,29.46 45.72,28.19 45.97,27.94 50.67,27.94 50.8,28.07 v51.31,28.07
  pour Top (no thermals): 38.99,27.81 39.62,27.81 39.62,28.7 40.39,29.46 42.04,29.46 42.04,30.1 39.62,30.1 39.62,29.59 38.99,28.96
N$69  (via drill 0.25)
  Top 0.152: NB16.2 63.75,22.48 64.39,21.84 v64.39,21.34 | v88.01,19.18 88.01,20.02 Q4.1
  Route2 0.152: v64.39,21.34 v64.39,17.4
  Route15 0.152: v64.39,17.4 82.17,17.4 83.95,19.18 v88.01,19.18
  pour Top (no thermals): 87.76,19.81 88.27,19.81 88.27,20.32 89.28,21.34 91.06,21.34 91.06,22.1 88.39,22.1 88.39,21.59 87.76,20.95
N$70
  Top 0.152: 32.68,52.07 C19.2
  Top 0.406: D2.C 29.97,52.2 30.1,52.07 C19.2
  pour Top (no thermals): 22.86,52.83 27.18,52.83 27.81,52.45 33.53,52.45 33.91,52.07 35.94,52.07 36.2,52.32 36.2,53.72 36.4,53.72 36.4,51.94 36.07,51.69 27.94,51.69 27.18,51.31 22.86,51.31
N$71
  Top 0.152: U4.2 35.81,52.58 35.69,52.45 34.29,52.45
  Top 0.203: 34.29,52.45 33.27,53.59 32.77,54.1 C19.1
N$73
